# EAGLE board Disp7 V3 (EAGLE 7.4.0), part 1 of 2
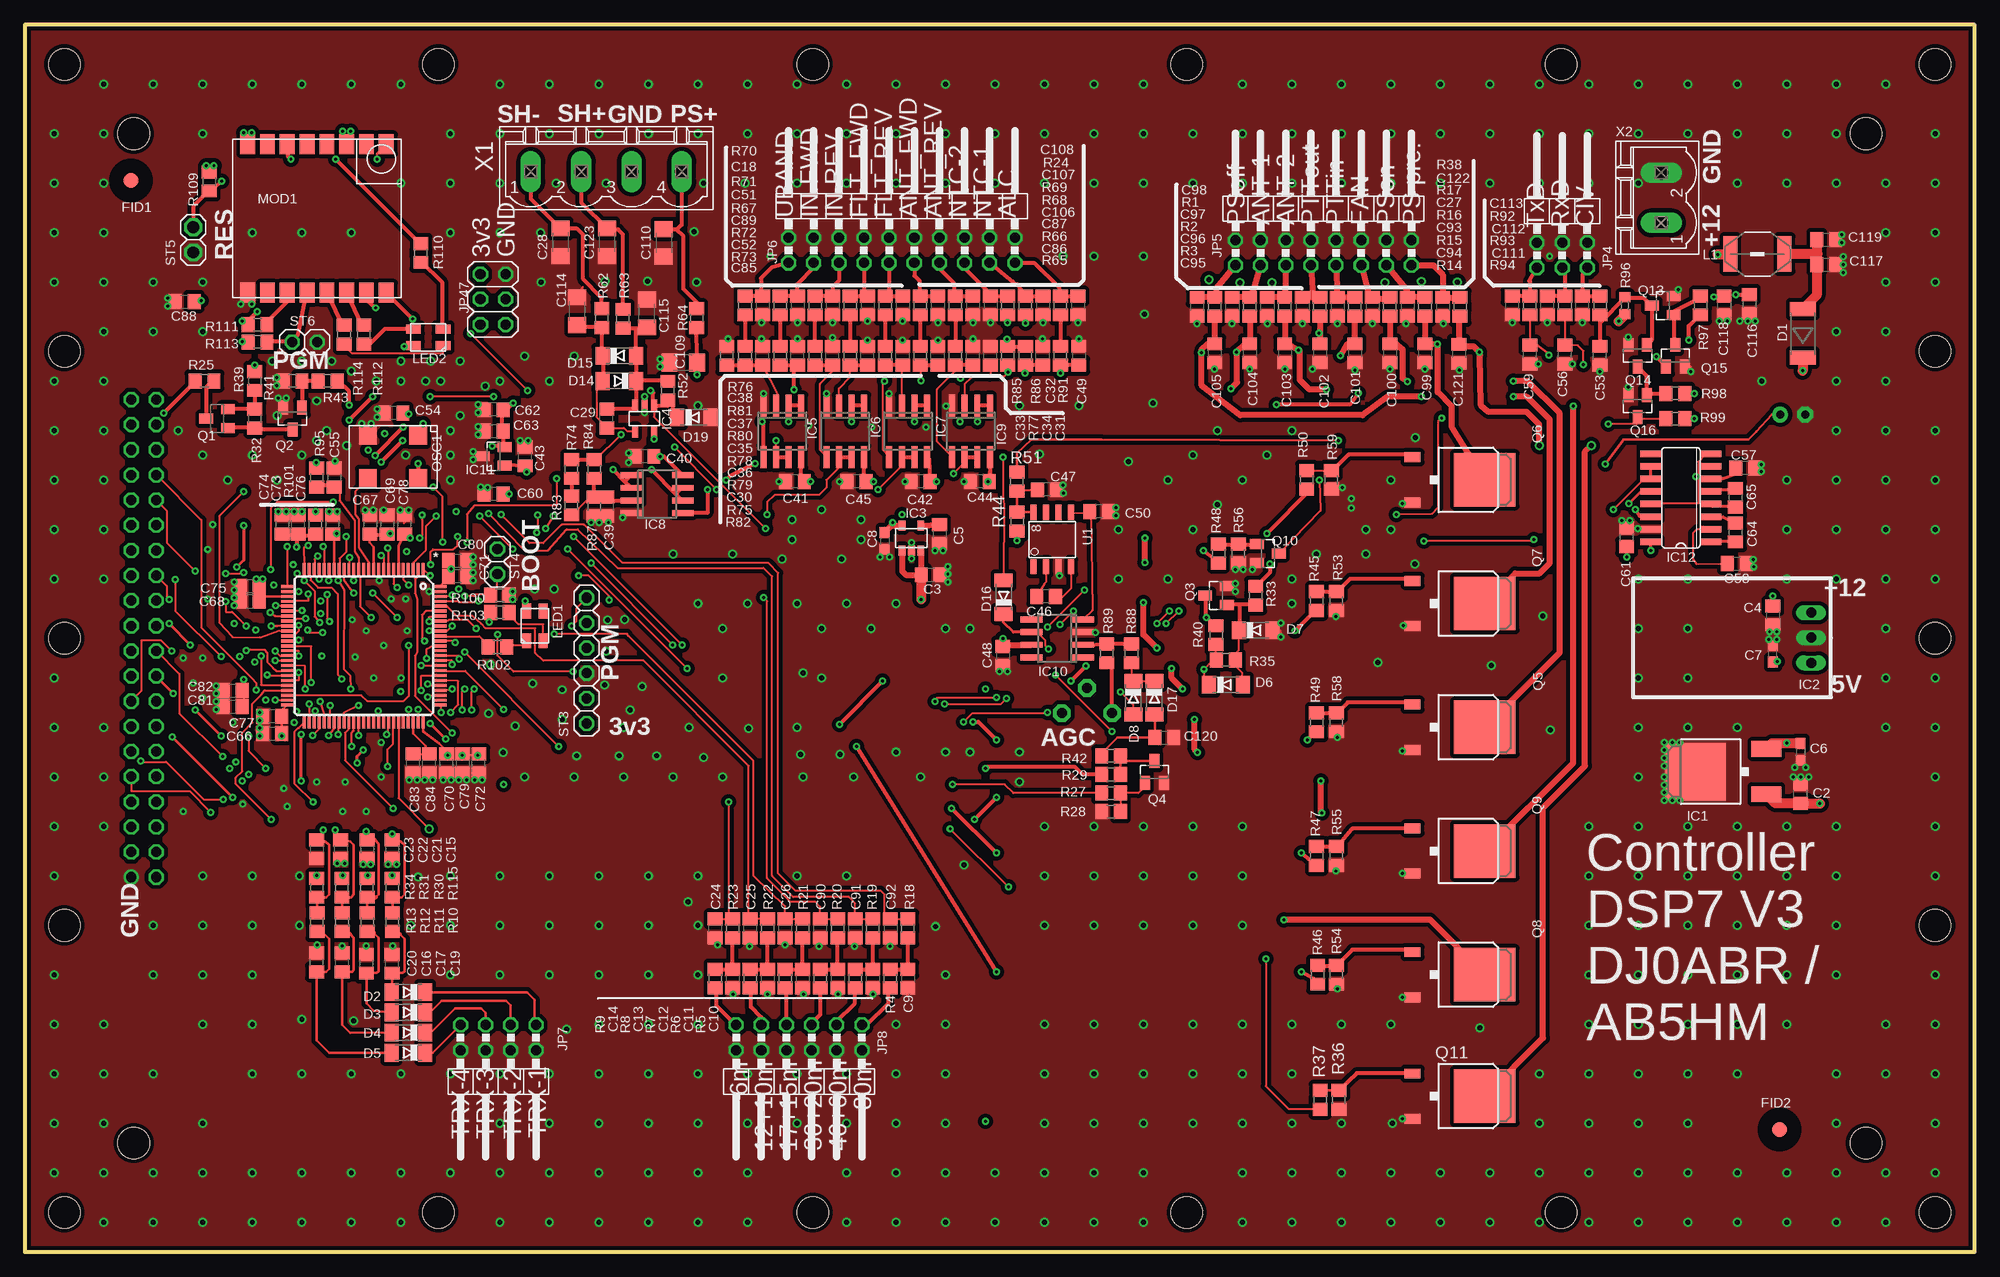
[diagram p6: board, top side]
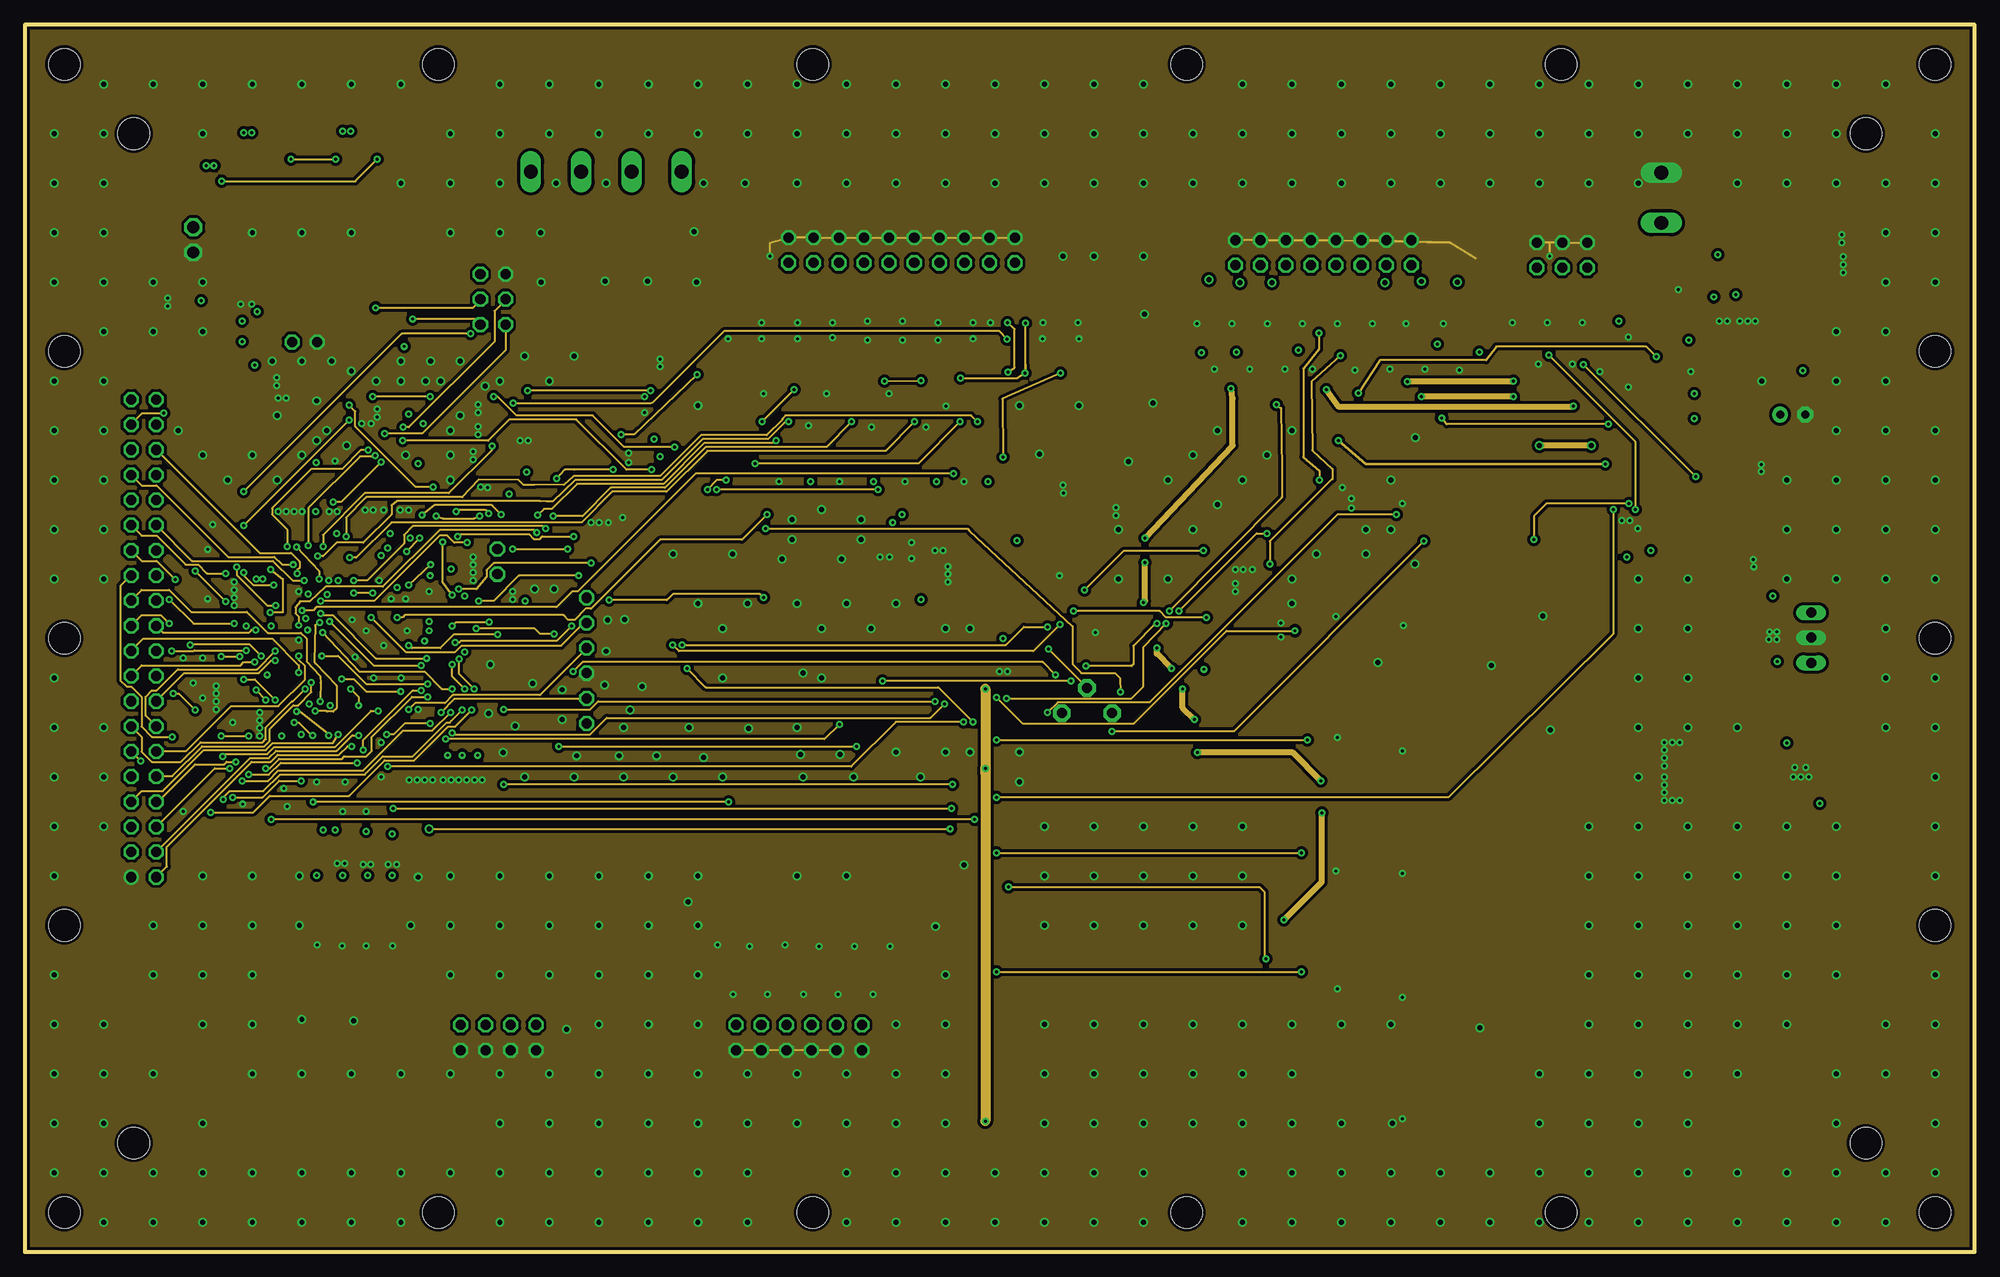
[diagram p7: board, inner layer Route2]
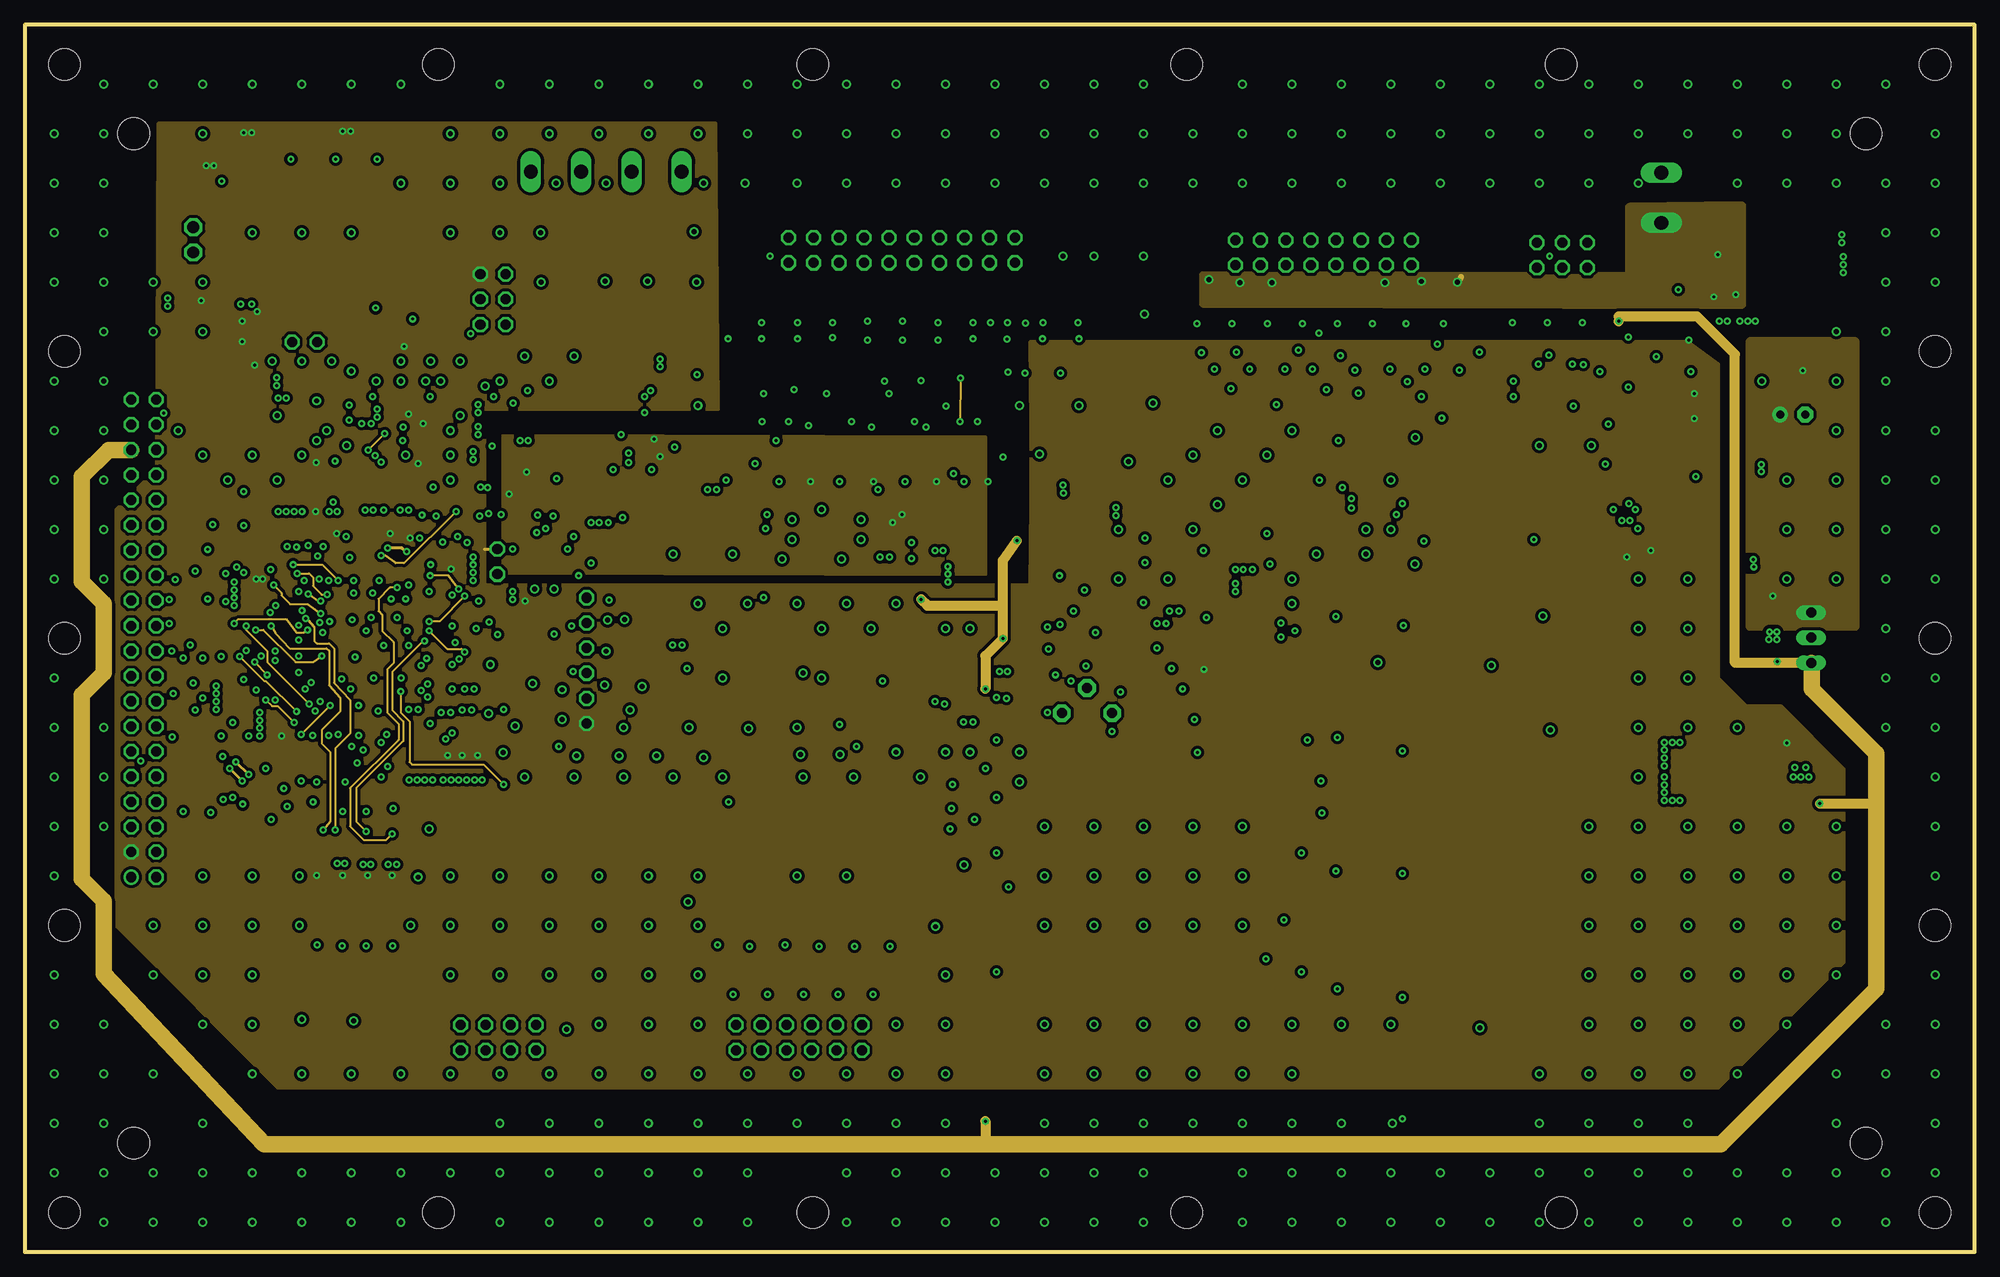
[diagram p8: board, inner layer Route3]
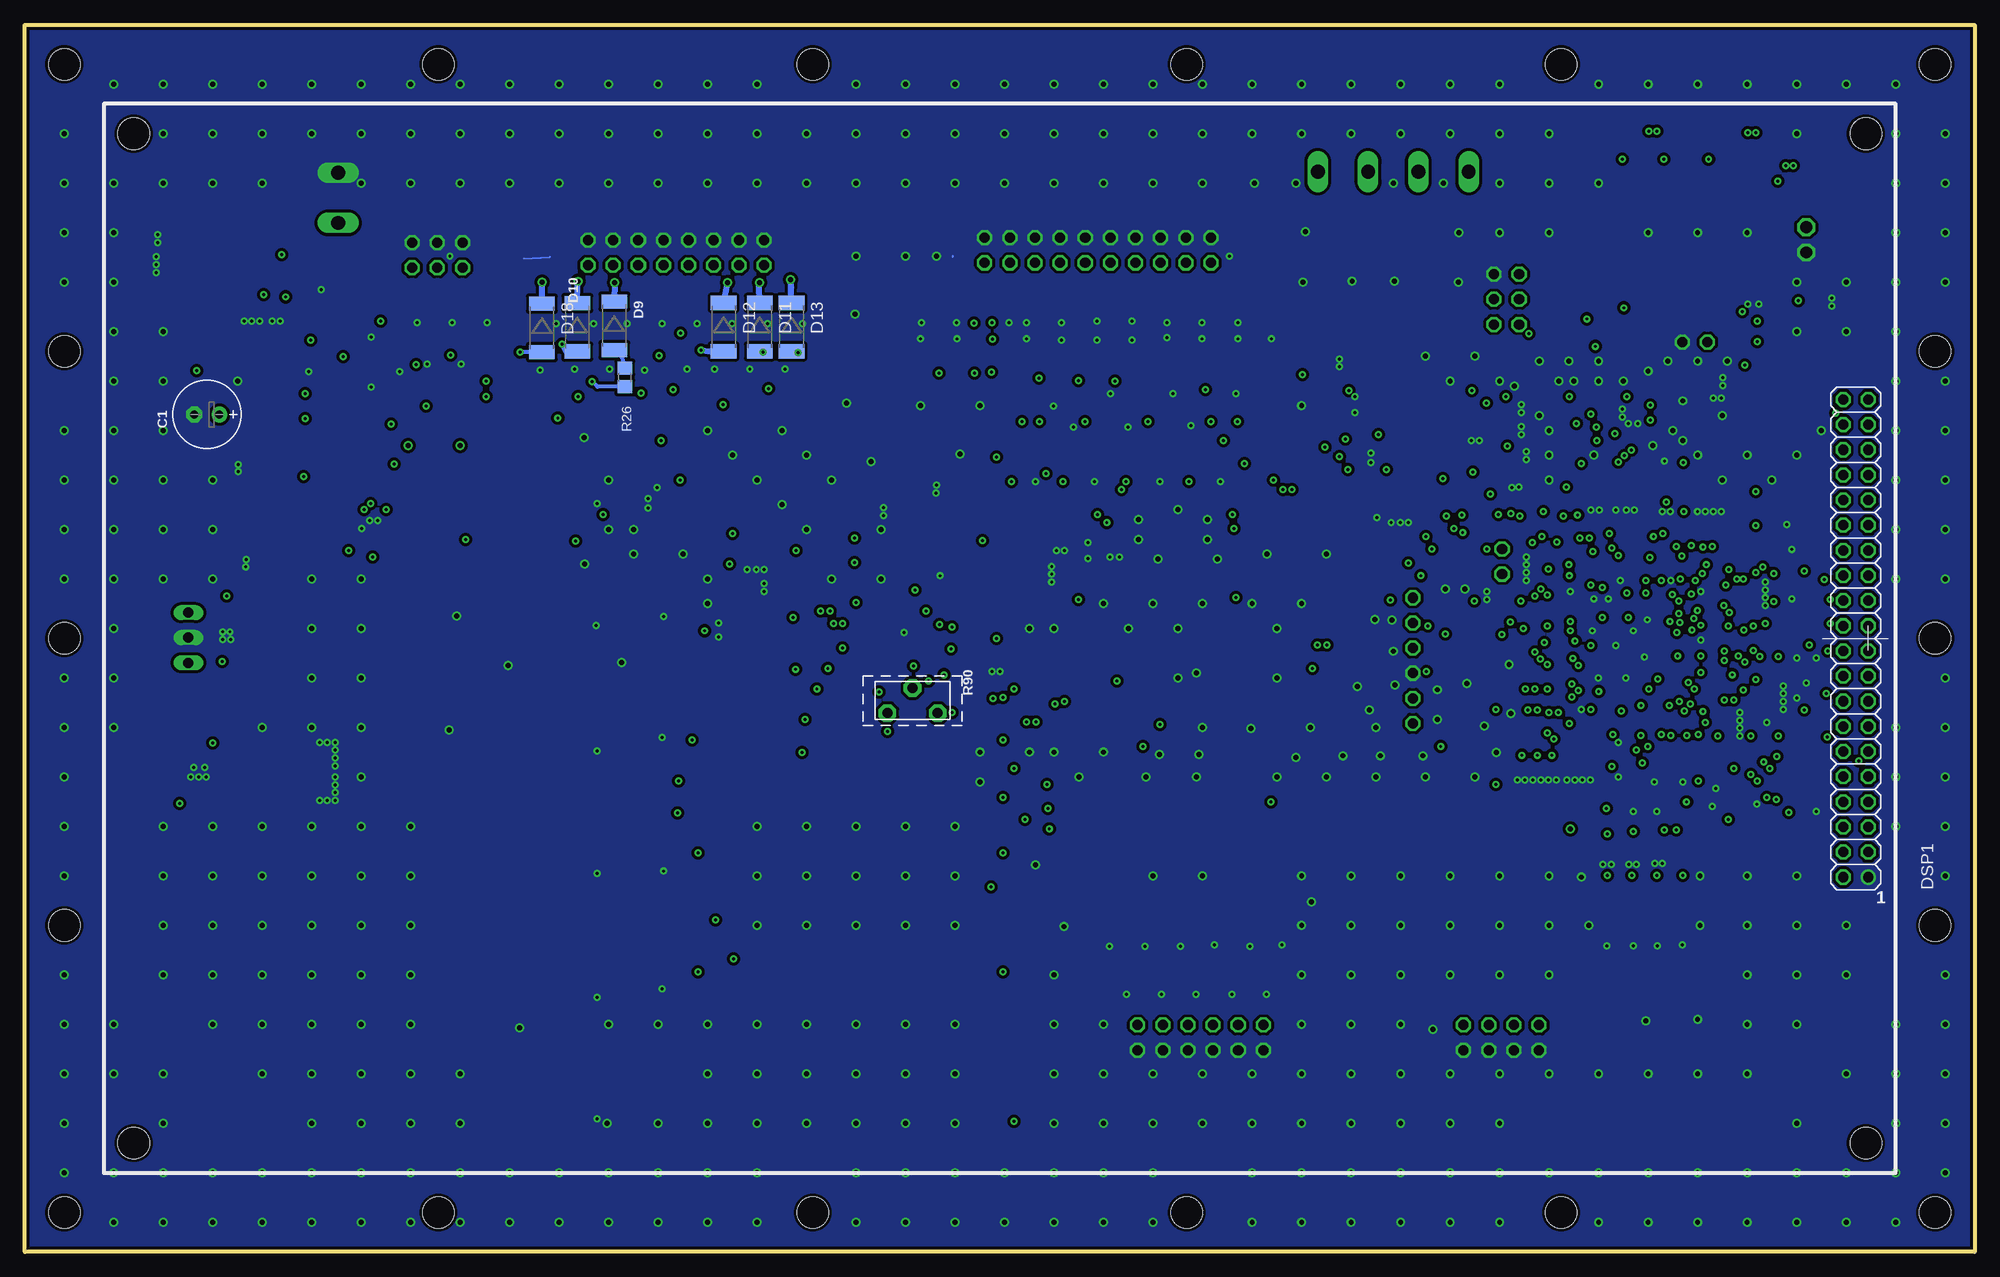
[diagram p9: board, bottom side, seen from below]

Size 197 x 124 mm. Coordinates in mm from the lower left corner, seen from the top.
Outline: 0,0 197,0 197,124 0,124 0,0
Copper layers (1+2*3+16): Top 0.035mm / dielectric 1.5mm / Route2 0.035mm / dielectric 0.15mm / Route3 0.035mm / dielectric 0.2mm / AGND$ 0.035mm
Design rules "default *": minimum track width 8mil, minimum drill 0.3mm, track to track 7mil, track to pad 7mil, pad to pad 7mil, via to via 7mil, smd to smd 0mil, copper to edge 10mil, drill to drill 8mil, minimum pad ring 10mil, minimum via ring 8mil, stop-mask expansion 0.02mm, vias tented up to drill 0.52mm, thermal gap 10mil
Net classes: 0 default: drill 0.3 mm; 1 Supply: width 0.203 mm, drill 0.3 mm, clearance 0.178 mm; 2 v12: drill 0.3 mm; 3 v533: drill 0.3 mm; 4 AGND: width 0.152 mm
Holes 3.2 mm at 4,120 193,120 193,4 4,4 4,91 4,62 4,33 193,91 193,62 193,33 41.8,120 79.6,120 117.4,120 155.2,120 41.8,4 79.6,4 117.4,4 155.2,4

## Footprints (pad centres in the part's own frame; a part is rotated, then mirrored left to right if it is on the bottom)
E2,5-7 = drill 0.813 pad 1.6: + -1.27,0 | drill 0.813 pad 1.6 octagon: - 1.27,0
C0805 = smd 1.3 x 1.5: 1 -0.95,0; 2 0.95,0
C0603 = smd 1.1 x 1: 1 -0.85,0; 2 0.85,0
C1206 = smd 1.6 x 1.8: 1 -1.4,0; 2 1.4,0
MELF = smd 1.45 x 2.6: 1 -2.445,0; 2 2.445,0
MINIMELF = smd 1.4 x 1.8: A 1.7,0; C -1.7,0
2X20 = drill 1.016: 1 2.747,78.13 | drill 1.016 octagon: 2 5.287,78.13; 3 2.747,75.59; 4 5.287,75.59; 5 2.747,73.05; 6 5.287,73.05; 7 2.747,70.51; 8 5.287,70.51; 9 2.747,67.97; 10 5.287,67.97; 11 2.747,65.43; 12 5.287,65.43; 13 2.747,62.89; 14 5.287,62.89; 15 2.747,60.35; 16 5.287,60.35; 17 2.747,57.81; 18 5.287,57.81; 19 2.747,55.27; 20 5.287,55.27; 21 2.747,52.73; 22 5.287,52.73; 23 2.747,50.19; 24 5.287,50.19; 25 2.747,47.65; 26 5.287,47.65; 27 2.747,45.11; 28 5.287,45.11; 29 2.747,42.57; 30 5.287,42.57; 31 2.747,40.03; 32 5.287,40.03; 33 2.747,37.49; 34 5.287,37.49; 35 2.747,34.95; 36 5.287,34.95; 37 2.747,32.41; 38 5.287,32.41; 39 2.747,29.87; 40 5.287,29.87 | hole 3.2: 3,105; 178,105; 178,3; 3,3
FIDUCIAL = smd 1.5 x 1.5: P$1 0,0
DPACK = smd 1.6 x 3: 1 -2.28,-4.8; 3 2.28,-4.8 | smd 5.8 x 6.2: 4 0,2.38
78SR_SWITCHREG = drill 1.016 long: 1 2.54,0; 2 0,0; 3 -2.54,0
SOT23-5 = smd 0.686 x 0.991: 1 -0.953,0; 2 0,0; 3 0.953,0; 4 0.953,2.54; 5 -0.953,2.54
SOT23-5' = smd 0.6 x 1.2: 1 -0.95,-1.306; 2 0,-1.306; 3 0.95,-1.306; 4 0.95,1.306; 5 -0.95,1.306
SO08 = smd 0.6 x 2.2: 1 -1.905,-2.6; 2 -0.635,-2.6; 3 0.635,-2.6; 4 1.905,-2.6; 5 1.905,2.6; 6 0.635,2.6; 7 -0.635,2.6; 8 -1.905,2.6
SOT23@1 = smd 1 x 1.4: 1 -0.95,-1.1; 2 0.95,-1.1; 3 0,1.1
SO16 = smd 0.66 x 2.032: 1 -4.445,-3.073; 2 -3.175,-3.073; 3 -1.905,-3.073; 4 -0.635,-3.073; 5 0.635,-3.073; 6 1.905,-3.073; 7 3.175,-3.073; 8 4.445,-3.073; 9 4.445,3.073; 10 3.175,3.073; 11 1.905,3.073; 12 0.635,3.073; 13 -0.635,3.073; 14 -1.905,3.073; 15 -3.175,3.073; 16 -4.445,3.073
TQFP100 = smd 1.2 x 0.3: 1 -7.75,6; 2 -7.75,5.5; 3 -7.75,5; 4 -7.75,4.5; 5 -7.75,4; 6 -7.75,3.5; 7 -7.75,3; 8 -7.75,2.5; 9 -7.75,2; 10 -7.75,1.5; 11 -7.75,1; 12 -7.75,0.5; 13 -7.75,0; 14 -7.75,-0.5; 15 -7.75,-1; 16 -7.75,-1.5; 17 -7.75,-2; 18 -7.75,-2.5; 19 -7.75,-3; 20 -7.75,-3.5; 21 -7.75,-4; 22 -7.75,-4.5; 23 -7.75,-5; 24 -7.75,-5.5; 25 -7.75,-6; 51 7.75,-6; 52 7.75,-5.5; 53 7.75,-5; 54 7.75,-4.5; 55 7.75,-4; 56 7.75,-3.5; 57 7.75,-3; 58 7.75,-2.5; 59 7.75,-2; 60 7.75,-1.5; 61 7.75,-1; 62 7.75,-0.5; 63 7.75,0; 64 7.75,0.5; 65 7.75,1; 66 7.75,1.5; 67 7.75,2; 68 7.75,2.5; 69 7.75,3; 70 7.75,3.5; 71 7.75,4; 72 7.75,4.5; 73 7.75,5; 74 7.75,5.5; 75 7.75,6 | smd 0.3 x 1.2: 26 -6,-7.75; 27 -5.5,-7.75; 28 -5,-7.75; 29 -4.5,-7.75; 30 -4,-7.75; 31 -3.5,-7.75; 32 -3,-7.75; 33 -2.5,-7.75; 34 -2,-7.75; 35 -1.5,-7.75; 36 -1,-7.75; 37 -0.5,-7.75; 38 0,-7.75; 39 0.5,-7.75; 40 1,-7.75; 41 1.5,-7.75; 42 2,-7.75; 43 2.5,-7.75; 44 3,-7.75; 45 3.5,-7.75; 46 4,-7.75; 47 4.5,-7.75; 48 5,-7.75; 49 5.5,-7.75; 50 6,-7.75; 76 6,7.75; 77 5.5,7.75; 78 5,7.75; 79 4.5,7.75; 80 4,7.75; 81 3.5,7.75; 82 3,7.75; 83 2.5,7.75; 84 2,7.75; 85 1.5,7.75; 86 1,7.75; 87 0.5,7.75; 88 0,7.75; 89 -0.5,7.75; 90 -1,7.75; 91 -1.5,7.75; 92 -2,7.75; 93 -2.5,7.75; 94 -3,7.75; 95 -3.5,7.75; 96 -4,7.75; 97 -4.5,7.75; 98 -5,7.75; 99 -5.5,7.75; 100 -6,7.75
2X03/90 = drill 1.016 octagon: 1 -2.54,-6.35; 2 -2.54,-3.81; 3 0,-6.35; 4 0,-3.81; 5 2.54,-6.35; 6 2.54,-3.81
2X08/90 = drill 1.016 octagon: 1 -8.89,-6.35; 2 -8.89,-3.81; 3 -6.35,-6.35; 4 -6.35,-3.81; 5 -3.81,-6.35; 6 -3.81,-3.81; 7 -1.27,-6.35; 8 -1.27,-3.81; 9 1.27,-6.35; 10 1.27,-3.81; 11 3.81,-6.35; 12 3.81,-3.81; 13 6.35,-6.35; 14 6.35,-3.81; 15 8.89,-6.35; 16 8.89,-3.81
2X10/90 = drill 1.016 octagon: 1 -11.43,-6.35; 2 -11.43,-3.81; 3 -8.89,-6.35; 4 -8.89,-3.81; 5 -6.35,-6.35; 6 -6.35,-3.81; 7 -3.81,-6.35; 8 -3.81,-3.81; 9 -1.27,-6.35; 10 -1.27,-3.81; 11 1.27,-6.35; 12 1.27,-3.81; 13 3.81,-6.35; 14 3.81,-3.81; 15 6.35,-6.35; 16 6.35,-3.81; 17 8.89,-6.35; 18 8.89,-3.81; 19 11.43,-6.35; 20 11.43,-3.81
2X04/90 = drill 1.016 octagon: 1 -3.81,-6.35; 2 -3.81,-3.81; 3 -1.27,-6.35; 4 -1.27,-3.81; 5 1.27,-6.35; 6 1.27,-3.81; 7 3.81,-6.35; 8 3.81,-3.81
2X06/90 = drill 1.016 octagon: 1 -6.35,-6.35; 2 -6.35,-3.81; 3 -3.81,-6.35; 4 -3.81,-3.81; 5 -1.27,-6.35; 6 -1.27,-3.81; 7 1.27,-6.35; 8 1.27,-3.81; 9 3.81,-6.35; 10 3.81,-3.81; 11 6.35,-6.35; 12 6.35,-3.81
2X03 = drill 1.016 octagon: 1 -2.54,-1.27; 2 -2.54,1.27; 3 0,-1.27; 4 0,1.27; 5 2.54,-1.27; 6 2.54,1.27
S = smd 1.4 x 3.56: 1 -2.73,0; 2 2.73,0
PLCC4_WE_LED = smd 1.5 x 0.9: 1 1.51,0.88; 2 1.51,-0.82; 3 -1.49,0.88; 4 -1.49,-0.82
ESP8266-12 = smd 1.5 x 2: P$1 0,0; P$2 2,0; P$3 4,0; P$4 6,0; P$5 8,0; P$6 10,0; P$7 12,0; P$8 14,0; P$9 14,15; P$10 12,15; P$11 10,15; P$12 8,15; P$13 6,15; P$14 4,15; P$15 2,15; P$16 0,15
QOSC_AQO7015 = smd 1.8 x 2: 1 0,-0.318; 2 5.08,-0.318; 3 5.08,4.128; 4 0,4.128
SOT23 = smd 1 x 1.4: 1 -0.95,-1.1; 2 0.95,-1.1; 3 0,1.1
D-PAK_TO252AA = smd 1 x 1.6: 1 -2.28,-4.8; 3 2.28,-4.8 | smd 5.4 x 6.2: 4 0,2.5
R0805 = smd 1.3 x 1.5: 1 -0.95,0; 2 0.95,0
MINIPOTI = drill 1.016 pad 1.778 octagon: 1 -2.54,-2.54; 2 2.54,-2.54; 3 0,0
R0603 = smd 1 x 1.1: 1 -0.85,0; 2 0.85,0
PINHEAD6X1 = drill 1.016 octagon: 1 -6.35,0; 2 -3.81,0; 3 -1.27,0; 4 1.27,0; 5 3.81,0; 6 6.35,0
PINHEAD1X2 = drill 1.016 octagon: 1 -1.27,0; 2 1.27,0
PINHEAD1X2BIG = drill 1.2 octagon: 1 -2.54,0; 2 0,0
SO-8 = smd 0.61 x 1.524: 1 -1.905,-2.743; 2 -0.635,-2.743; 3 0.635,-2.743; 4 1.905,-2.743; 5 1.905,2.743; 6 0.635,2.743; 7 -0.635,2.743; 8 -1.905,2.743
MSTBV4 = drill 1.397 long: 1 -7.62,0; 2 -2.54,0; 3 2.54,0; 4 7.62,0
MSTBV2 = drill 1.397 long: 1 -2.54,0; 2 2.54,0

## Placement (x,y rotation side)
C1  100u/16  [E2,5-7]  178.61,84.63 180 bottom
C2  10u  [C0805]  179.4,46.29 90 top
C3  10u  [C0805]  91.52,68.42 0 top
C4  10u  [C0805]  176.6,64.32 270 top
C5  10n  [C0805]  92.42,72.54 270 top
C6  10u  [C0603]  179.4,50.54 270 top
C7  10u  [C0603]  176.6,60.45 90 top
C8  10u  [C0603]  86.88,71.86 270 top
C9  100n  [C0805]  89.22,27.62 270 top
C10  100n  [C0805]  85.67,27.62 270 top
C11  100n  [C0805]  82.14,27.62 270 top
C12  100n  [C0805]  78.59,27.62 270 top
C13  100n  [C0805]  75.06,27.62 270 top
C14  100n  [C0805]  71.52,27.62 270 top
C15  100n  [C0805]  37.12,40.7 270 top
C16  100n  [C0805]  32.06,29.25 90 top
C17  100n  [C0805]  34.52,29.13 90 top
C18  100n  [C0805]  74.54,95.63 270 top
C19  100n  [C0805]  37.1,29.13 90 top
C20  100n  [C0805]  29.48,29.25 90 top
C21  100n  [C0805]  34.59,40.7 270 top
C22  100n  [C0805]  31.92,40.7 270 top
C23  100n  [C0805]  29.5,40.7 270 top
C24  100n  [C0805]  69.75,32.7 270 top
C25  100n  [C0805]  73.28,32.7 270 top
C26  100n  [C0805]  76.83,32.7 270 top
C27  100n  [C0805]  139.68,95.5 270 top
C28  100n/200V  [C1206]  54.12,102.02 270 top
C29  10u  [C0805]  58.8,84.2 90 top
C30  100n  [C0805]  74.54,90.55 90 top
C31  1u  [C0805]  97.57,90.55 90 top
C32  1u  [C0805]  102.84,90.55 90 top
C33  10n  [C0805]  92.24,90.55 90 top
C34  10n  [C0805]  95.78,90.55 90 top
C35  10n  [C0805]  81.62,90.55 90 top
C36  10n  [C0805]  78.08,90.55 90 top
C37  10n  [C0805]  85.16,90.55 90 top
C38  10n  [C0805]  88.7,90.55 90 top
C39  1u  [C0805]  58.8,75.31 270 top
C40  1u  [C0805]  62.61,80.39 180 top
C41  1u  [C0805]  77.81,77.85 180 top
C42  1u  [C0805]  90.51,77.85 180 top
C43  1u  [C0805]  50.55,80.39 90 top
C44  1u  [C0805]  96.48,77.85 180 top
C45  1u  [C0805]  84.03,77.85 180 top
C46  10u  [C0805]  103.19,66.24 180 top
C47  1u  [C0805]  103.27,77.02 180 top
C48  1u  [C0805]  98.81,60.24 270 top
C49  10n  [C0805]  106.48,90.55 270 top
C50  10u  [C0805]  108.54,74.81 180 top
C51  10n  [C0805]  78.08,95.63 270 top
C52  10n  [C0805]  85.16,95.63 270 top
C53  1n  [C0805]  159.13,90.55 90 top
C54  1u  [C0805]  37.25,84.75 180 top
C55  100n  [C0805]  31.25,78.25 270 top
C56  1n  [C0805]  155.59,90.67 90 top
C57  1u  [C0805]  173.82,79.21 180 top
C58  1u  [C0805]  172.96,69.56 0 top
C59  1n  [C0805]  152.05,90.67 90 top
C60  100n  [C0805]  47.37,76.58 180 top
C61  1u  [C0805]  161.82,72.21 270 top
C62  100n  [C0805]  47.37,85.09 180 top
C63  1u  [C0805]  47.37,82.93 0 top
C64  1u  [C0805]  172.82,72.71 270 top
C65  1u  [C0805]  172.82,76.21 270 top
C66  4u7  [C0805]  25,52.38 0 top
C67  100n  [C0805]  34.88,73.5 270 top
C68  100n  [C0805]  22.75,65.75 0 top
C69  100n  [C0805]  36.62,73.5 270 top
C70  100n  [C0805]  42.62,49.38 90 top
C71  100n  [C0805]  43.75,68.25 180 top
C72  100n  [C0805]  45.88,49.38 90 top
C73  100n  [C0805]  27.62,73.5 90 top
C74  1u  [C0805]  26,73.5 270 top
C75  100n  [C0805]  22.75,67.25 180 top
C76  100n  [C0805]  31.12,73.5 90 top
C77  100n  [C0805]  25,54.12 180 top
C78  100n  [C0805]  38.38,73.5 90 top
C79  100n  [C0805]  44.25,49.38 270 top
C80  100n  [C0805]  43.75,69.88 0 top
C81  1u  [C0805]  21,55.12 0 top
C82  1u  [C0805]  21,56.75 0 top
C83  1u  [C0805]  39.25,49.38 90 top
C84  1u  [C0805]  40.88,49.38 90 top
C85  10n  [C0805]  88.7,95.63 270 top
C86  10n  [C0805]  92.24,95.63 270 top
C87  10n  [C0805]  95.78,95.63 270 top
C88  10u  [C0805]  16.16,96.04 0 top
C89  10n  [C0805]  81.62,95.63 270 top
C90  100n  [C0805]  80.36,32.7 270 top
C91  100n  [C0805]  83.91,32.7 270 top
C92  100n  [C0805]  87.44,32.7 270 top
C93  100n  [C0805]  136.14,95.5 270 top
C94  100n  [C0805]  132.6,95.5 270 top
C95  100n  [C0805]  129.06,95.5 270 top
C96  100n  [C0805]  125.52,95.5 270 top
C97  100n  [C0805]  121.98,95.5 270 top
C98  100n  [C0805]  118.44,95.5 270 top
C99  100n  [C0805]  141.45,90.8 270 top
C100  100n  [C0805]  137.91,90.8 270 top
C101  100n  [C0805]  134.37,90.8 270 top
C102  100n  [C0805]  130.83,90.8 270 top
C103  100n  [C0805]  127.29,90.8 270 top
C104  100n  [C0805]  123.75,90.8 270 top
C105  100n  [C0805]  120.21,90.8 270 top
C106  100n  [C0805]  97.57,95.63 270 top
C107  100n  [C0805]  102.86,95.63 270 top
C108  100n  [C0805]  106.4,95.63 270 top
C109  100n/200V  [C1206]  66.52,89.85 180 top
C110  100n/200V  [C1206]  64.55,101.95 270 top
C111  1n  [C0805]  157.36,95.63 90 top
C112  1n  [C0805]  153.82,95.63 90 top
C113  1n  [C0805]  150.28,95.63 90 top
C114  100n/200V  [C1206]  55.81,95.06 90 top
C115  100n/200V  [C1206]  62.87,94.82 90 top
C116  10u  [C0805]  174.21,95.79 270 top
C117  10u  [C0805]  181.99,99.76 0 top
C118  100n  [C0805]  171.67,95.63 270 top
C119  100n  [C0805]  181.99,102.3 0 top
C120  10n  [C0805]  115.12,52 0 top
C121  100n  [C0805]  144.88,90.75 270 top
C122  100n  [C0805]  143.25,95.5 270 top
C123  100n/200V  [C1206]  58.83,102.03 270 top
D1  1N4001  [MELF]  179.62,92.81 90 top
D2  1N4448  [MINIMELF]  38.76,26.25 180 top
D3  1N4448  [MINIMELF]  38.76,24.21 180 top
D4  1N4448  [MINIMELF]  38.76,22.17 180 top
D5  1N4448  [MINIMELF]  38.76,20.13 180 top
D6  NTS245SFT1G  [MINIMELF]  121.35,57.32 0 top
D7  NTS245SFT1G  [MINIMELF]  124.35,62.82 0 top
D8  1N4448  [MINIMELF]  112,56 270 top
D9  SS110B  [MELF]  137.44,93.58 270 bottom
D10  SS110B  [MELF]  141.18,93.43 270 bottom
D11  SS110B  [MELF]  122.75,93.45 270 bottom
D12  SS110B  [MELF]  126.39,93.45 270 bottom
D13  SS110B  [MELF]  119.54,93.45 270 bottom
D14  NTS245SFT1G  [MINIMELF]  60.07,88.01 180 top
D15  NTS245SFT1G  [MINIMELF]  60.07,90.55 0 top
D16  1N4448  [MINIMELF]  98.88,66.16 90 top
D17  1N4448  [MINIMELF]  114.12,56 270 top
D18  SS110B  [MELF]  144.75,93.38 270 bottom
D19  *3V  [MINIMELF]  67.6,84.33 0 top
DSP1  DISPLAY7DISPL7_ARDUINO  [2X20]  8,116 180 bottom
FID1  FIDUCIAL  [FIDUCIAL]  10.73,108.26 0 top
FID2  FIDUCIAL  [FIDUCIAL]  177.29,12.37 0 top
IC1  LF33CDT-DPAK  [DPACK]  171.15,48.54 90 top
IC2  7805 (7962138)  [78SR_SWITCHREG]  180.48,62.07 90 top
IC3  LP2992 3v3  [SOT23-5]  89.58,70.87 0 top
IC4  INA193AQDBVRQ1  [SOT23-5']  62.61,84.2 180 top
IC5  TS27L2C  [SO08]  76.54,82.93 180 top
IC6  TS27L2C  [SO08]  82.89,82.93 180 top
IC7  TS27L2C  [SO08]  89.24,82.93 180 top
IC8  TS27L2C  [SO08]  63.88,76.58 270 top
IC9  TS27L2C  [SO08]  95.59,82.93 180 top
IC10  TL081D  [SO08]  104.31,61.99 90 top
IC11  ADR381  [SOT23@1]  47.37,80.39 90 top
IC12  MAX3232  [SO16]  167.32,76.21 90 top
IC13  STM32F427VGT6  [TQFP100]  34.25,61.25 270 top
JP4  [2X03/90]  155.32,105.79 0 top
JP5  [2X08/90]  131.2,106.04 0 top
JP6  [2X10/90]  88.59,106.29 0 top
JP7  TRX Detector  [2X04/90]  47.84,16.59 180 top
JP8  Band Relais  [2X06/90]  78.22,16.59 180 top
JP47  [2X03]  47.3,96.26 270 top
L1  WE74451147/47uH  [S]  175.05,100.84 180 top
LED1  RGBLED  [PLCC4_WE_LED]  51.57,63.25 90 top
LED2  RGBLED  [PLCC4_WE_LED]  40.77,92.44 180 top
MOD1  ESP-07S (ESP8266)  [ESP8266-12]  22.52,96.94 0 top
OSC1  OSZ8MHz  [QOSC_AQO7015]  39.75,82.25 180 top
Q1  IRLML6401  [SOT23]  19.43,84.2 90 top
Q2  N-CH_MOSFET  [SOT23]  27.05,84.2 180 top
Q3  N-CH_MOSFET  [SOT23]  120.35,66.32 90 top
Q4  BS170_SMD  [SOT23]  114.12,48.5 0 top
Q5  IRLR120N  [D-PAK_TO252AA]  145,53.02 270 top
Q6  IRLR120N  [D-PAK_TO252AA]  145,78.02 270 top
Q7  IRLR120N  [D-PAK_TO252AA]  145,65.52 270 top
Q8  IRLR120N  [D-PAK_TO252AA]  145,28.02 270 top
Q9  IRLR120N  [D-PAK_TO252AA]  145,40.52 270 top
Q10  N-CH_MOSFET  [SOT23]  125.6,70.57 270 top
Q11  IRLR120N  [D-PAK_TO252AA]  145,15.75 270 top
Q13  N-CH_MOSFET  [SOT23]  165.48,95.63 90 top
Q14  N-CH_MOSFET  [SOT23]  162.94,90.55 180 top
Q15  N-CH_MOSFET  [SOT23]  166.75,90.55 0 top
Q16  N-CH_MOSFET  [SOT23]  162.94,85.47 180 top
R1  1kOhm-Ferrit  [R0805]  120.21,95.5 270 top
R2  1kOhm-Ferrit  [R0805]  123.75,95.5 270 top
R3  1kOhm-Ferrit  [R0805]  127.29,95.5 270 top
R4  100  [R0805]  87.44,27.62 90 top
R5  100  [R0805]  83.91,27.62 90 top
R6  100  [R0805]  80.36,27.62 90 top
R7  100  [R0805]  76.83,27.62 90 top
R8  100  [R0805]  73.28,27.62 90 top
R9  100  [R0805]  69.75,27.62 90 top
R10  1kOhm-Ferrit  [R0805]  37.15,33.33 90 top
R11  1kOhm-Ferrit  [R0805]  34.61,33.33 90 top
R12  1kOhm-Ferrit  [R0805]  32.06,33.33 90 top
R13  1kOhm-Ferrit  [R0805]  29.52,33.33 90 top
R14  1kOhm-Ferrit  [R0805]  130.83,95.5 270 top
R15  1kOhm-Ferrit  [R0805]  134.37,95.5 270 top
R16  1kOhm-Ferrit  [R0805]  137.91,95.5 270 top
R17  1kOhm-Ferrit  [R0805]  141.45,95.5 270 top
R18  1kOhm-Ferrit  [R0805]  89.22,32.7 270 top
R19  1kOhm-Ferrit  [R0805]  85.67,32.7 270 top
R20  1kOhm-Ferrit  [R0805]  82.14,32.7 270 top
R21  1kOhm-Ferrit  [R0805]  78.59,32.7 270 top
R22  1kOhm-Ferrit  [R0805]  75.06,32.7 270 top
R23  1kOhm-Ferrit  [R0805]  71.52,32.7 270 top
R24  1kOhm-Ferrit  [R0805]  104.63,95.63 90 top
R25  220  [R0805]  18.16,88.01 0 top
R26  ***  [R0805]  136.38,88.38 270 bottom
R27  1k  [R0805]  109.75,46.38 0 top
R28  100k  [R0805]  109.75,44.5 0 top
R29  1k  [R0805]  109.75,48.25 180 top
R30  10k  [R0805]  34.59,36.8 90 top
R31  10k  [R0805]  32.05,36.8 90 top
R32  1k  [R0805]  23.24,84.2 270 top
R33  1k  [R0805]  124.35,66.32 270 top
R34  10k  [R0805]  29.5,36.8 90 top
R35  1M  [R0805]  121.35,59.82 0 top
R36  100k  [R0805]  132.75,15.38 270 top
R37  1k  [R0805]  130.88,15.38 90 top
R38  1kOhm-Ferrit  [R0805]  145,95.5 270 top
R39  100  [R0805]  23.24,88.01 90 top
R40  100k  [R0805]  120.35,62.32 270 top
R41  100k  [R0805]  27.05,88.01 180 top
R42  10k  [R0805]  109.75,50.12 0 top
R43  1k  [R0805]  30.61,88.01 180 top
R44  oR  [R0805]  100.25,73.8 90 top
R45  1k  [R0805]  130.5,65.77 90 top
R46  1k  [R0805]  130.62,28.02 90 top
R47  1k  [R0805]  130.5,40.02 90 top
R48  1k  [R0805]  120.6,70.57 90 top
R49  1k  [R0805]  130.5,53.52 90 top
R50  1k  [R0805]  129.5,78.02 90 top
R51  ***  [R0805]  100.22,77.85 270 top
R52  *10k  [R0805]  64.97,87.03 270 top
R53  100k  [R0805]  132.5,65.77 270 top
R54  100k  [R0805]  132.5,28.02 270 top
R55  100k  [R0805]  132.5,40.02 270 top
R56  100k  [R0805]  122.6,70.57 270 top
R58  100k  [R0805]  132.5,53.52 270 top
R59  100k  [R0805]  132,78.02 270 top
R62  1kOhm-Ferrit  [R0805]  58.3,94.36 270 top
R63  1kOhm-Ferrit  [R0805]  60.44,94.28 270 top
R64  1kOhm-Ferrit  [R0805]  67.88,94.36 270 top
R65  1kOhm-Ferrit  [R0805]  90.47,95.63 270 top
R66  1kOhm-Ferrit  [R0805]  94.01,95.63 270 top
R67  1kOhm-Ferrit  [R0805]  79.85,95.63 270 top
R68  1kOhm-Ferrit  [R0805]  99.3,95.63 270 top
R69  1kOhm-Ferrit  [R0805]  101.09,95.63 270 top
R70  1kOhm-Ferrit  [R0805]  72.77,95.63 270 top
R71  1kOhm-Ferrit  [R0805]  76.31,95.63 270 top
R72  1kOhm-Ferrit  [R0805]  83.39,95.63 270 top
R73  1kOhm-Ferrit  [R0805]  86.93,95.63 270 top
R74  NC  [R0805]  55.24,79.12 90 top
R75  22k  [R0805]  72.77,90.55 90 top
R76  1k  [R0805]  90.47,90.55 90 top
R77  1k  [R0805]  94.01,90.55 90 top
R78  1k  [R0805]  79.85,90.55 90 top
R79  1k  [R0805]  76.31,90.55 90 top
R80  1k  [R0805]  83.39,90.55 90 top
R81  1k  [R0805]  86.93,90.55 90 top
R82  10k  [R0805]  70.93,90.55 270 top
R83  390k/0,1%  [R0805]  55.24,75.44 90 top
R84  390k/0,1%  [R0805]  57.53,79.12 90 top
R85  8k2  [R0805]  99.3,90.55 270 top
R86  8k2  [R0805]  101.09,90.55 270 top
R87  10k/0,1%  [R0805]  57.53,75.31 90 top
R88  10k  [R0805]  111.81,60.49 90 top
R89  1k  [R0805]  109.31,60.49 90 top
R90  50k  [MINIPOTI]  107.31,56.99 0 bottom
R91  100  [R0805]  104.63,90.55 90 top
R92  1kOhm-Ferrit  [R0805]  152.05,95.63 270 top
R93  1kOhm-Ferrit  [R0805]  155.59,95.63 270 top
R94  1kOhm-Ferrit  [R0805]  159.13,95.63 270 top
R95  100k  [R0805]  29.5,78.25 270 top
R96  10k  [R0603]  161.67,95.63 270 top
R97  10k  [R0805]  169.29,95.63 270 top
R98  10k  [R0805]  166.75,86.74 0 top
R99  10k  [R0805]  166.75,84.2 0 top
R100  10k  [R0805]  48,66.38 180 top
R101  1kOhm-Ferrit  [R0805]  29.38,73.5 270 top
R102  2k2  [R0805]  47.75,61.12 180 top
R103  680  [R0805]  48,64.62 180 top
R109  100k  [R0805]  18.64,108.16 90 top
R110  1k  [R0805]  40.02,100.94 90 top
R111  100k  [R0805]  23.52,93.69 180 top
R112  1k  [R0805]  34.27,92.69 90 top
R113  100k  [R0805]  23.52,91.94 180 top
R114  1k  [R0805]  32.27,92.69 90 top
R115  10k  [R0805]  37.12,36.8 90 top
ST3  SWD  [PINHEAD6X1]  56.75,59.75 90 top
ST4  [PINHEAD1X2]  47.75,69.75 270 top
ST5  [PINHEAD1X2BIG]  17.03,103.54 90 top
ST6  PGM  [PINHEAD1X2]  28.27,91.94 180 top
U1  TC7662AEPASOIC  [SO-8]  103.81,71.99 0 top
X1  MSTBV4  [MSTBV4]  58.75,109.15 0 top
X2  MSTBV2  [MSTBV2]  165.32,106.53 90 top

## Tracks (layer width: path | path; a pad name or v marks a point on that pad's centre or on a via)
+5V  (via drill 0.3)
  Top 0.203: 176.45,59.7 C7.1 | v98.81,61.98 98.96,61.82 98.96,61.66 99.08,61.35
  Top 0.254: 100.27,72.83 R44.1 v100.22,71.88
  Top 0.305: v177.04,59.66 176.45,59.7
  Top 0.406: R29.2 106.88,48.25 106.12,49 97.18,49 v97.06,48.88
  Top 0.61: IC3.3 90.57,70.83 C3.1 89.02,68.42 88.64,68.8 88.64,70.85 IC3.1 | 98.81,61.09 C48.1 99.08,61.35 IC10.7
  Top 1.016: IC1.1 176.87,45.34 C2.1 179.43,45.31 v181.35,45.31 | v161.03,94.04 161.67,94.68 R96.2 | C3.1 90.55,68.41 v90.55,65.94
  Route2 0.406: 97.06,13.24 97,13.24 v97.08,13.22
  Route2 1.016: v97.06,56.9 v97.06,48.88 | 97.06,48.38 v97.06,48.88 | v97.06,48.88 97.06,13.24
  Route3 0.406: v97.08,13.22 97.06,13.22 | v177.04,59.66 180.48,59.66 IC2.3
  Route3 1.016: IC2.3 172.78,59.53 172.78,90.71 168.97,94.52 161.03,94.52 v161.03,94.04 | 98.81,65.31 v98.81,61.98 97.06,60.23 v97.06,56.9 | 98.81,65.31 98.81,69.88 v100.22,71.88 | v181.35,45.31 187.07,45.31 | v90.55,65.94 91.19,65.31 98.81,65.31 | 97.06,13.24 97.06,13.22 97.06,10.86
  Route3 1.676: IC2.3 180.56,59.45 180.56,56.9 187.07,50.39 187.07,45.31 187.07,26.57 171.35,10.86 97.06,10.86 24.19,10.86 8,28.08 8,35.46 5.78,37.69 5.78,56.26 8,58.48 8,65.5 5.78,67.72 5.78,78.33 8.5,81.05 DSP1.35
+UB  (via drill 0.3)
  Top 0.203: 176.58,65.32 C4.1 | 179.61,90.31 D1.1
  Top 0.254: v159.7,79.6 161.43,82 161.5,82.08 174.1,82.08 174.93,82.9 176.5,84.62 C1.+ | v132.7,82 108.78,82.08 101.72,82.08 100.22,80.72 R51.1
  Top 0.305: v176.58,66.26 176.58,65.32
  Top 1.016: 179.61,90.31 v179.61,89.04
  Route2 0.254: v159.7,79.6 135.47,79.6 v132.7,82
  pour Route3 (isolate 0.305, no thermals): 174.37,91.98 184.85,91.98 184.85,63.24 174.37,63.24
/CS  (via drill 0.3)
  Top 0.203: v40.62,59.99 40.62,60.93 41.26,61.26 IC13.88 | v22.13,68.64 21.81,68.64 21.73,68.56 v20.3,68.56
  Route2 0.203: v40.62,59.99 35.46,59.99 31.1,64.36 30.15,64.36 v29.91,64.49 | v25.14,67.37 23.08,67.37 22.13,68.33 v22.13,68.64 | v20.3,68.56 18.4,68.56 17.52,69.44 16.26,69.44 13.32,72.37 11.81,72.37 10.78,73.41 DSP1.29
  Route3 0.203: v29.91,64.49 28.56,65.47 26.81,65.47 25.94,66.34 25.94,66.58 v25.14,67.37
/RD  (via drill 0.3)
  Top 0.203: v43.16,59.36 43.16,59.75 42.05,59.75 IC13.85 | v44.43,56.9 44.2,56.66 v44.2,54.75 | v20.07,45.7 18.08,45.7 14.27,49.51 11.73,49.51 v11.73,49.59
  Route2 0.203: v43.16,59.36 43.16,58.16 v44.43,56.9 | v44.2,54.75 42.92,53.48 42.61,53.48 39.19,50.07 36.18,50.07 34.35,48.24 25.78,48.24 24.11,46.58 20.7,46.58 20.07,45.94 v20.07,45.7 | v11.73,49.59 10.78,50.55 DSP1.11
/RES  (via drill 0.3)
  Top 0.203: v33.71,55.22 32.25,54.5 32.21,54.46 32.21,53.56 IC13.59 | v31.65,67.85 32.25,66.88 32.22,58.9 32.88,58.25 v32.9,56.9
  Route2 0.203: v33.71,55.22 33.71,56.1 v32.9,56.9 | v27.13,69.44 26.02,69.44 25.22,70.23 20.54,70.23 13.32,77.45 11.81,77.45 10.78,78.48 DSP1.33
  Route3 0.203: v31.65,67.85 30.07,69.44 v27.13,69.44
/RW  (via drill 0.3)
  Top 0.203: v43.88,59.91 43.88,60.23 42.05,60.23 IC13.86 | v45.39,56.9 45.15,56.66 v45.15,54.75 | v18.8,44.43 16.65,46.58 10.78,46.58 10.78,48.01 DSP1.9
  Route2 0.203: v43.88,59.91 43.88,58.4 v45.39,56.9 | v45.15,54.75 43.48,53.09 42.77,53.09 39.35,49.67 36.34,49.67 32.77,46.1 24.75,46.1 23.08,44.43 v18.8,44.43
AGC  (via drill 0.3)
  Top 0.203: IC13.24 28.75,68.38 28.88,68.12 28.88,67.88 29.62,67.12 31,67.12 31.62,66.5 31.62,58.38 v32,57.88 | R27.1 99.88,46.38 99,47.25 v93.75,47.25
  Route2 0.203: v93.75,47.25 v48.38,47.25 | v32,57.88 33.25,57.88 34.5,56.62 v38,56.62
  Route3 0.203: v38,56.62 38,54.5 38.88,53.62 38.88,49.5 39.12,49.25 46.38,49.25 v48.38,47.25
AGND  (via drill 0.3, 0.5)
  Top 0.203: v19.34,55.62 19.59,55.31 20.3,55.31 C81.1 | v19.34,56.42 19.34,56.74 20.3,56.74 C82.1 | v35.62,84.36 35.62,84.68 36.34,84.68 C54.2 | v39.63,47.69 39.25,48.21 39.02,48.45 C83.1 | v41.22,47.69 40.84,48.13 40.52,48.45 C84.1 | v174.66,69.23 173.79,69.21 173.85,69.27 C58.2 | v175.45,79.58 175.2,79.27 174.89,79.27 C57.1 | v23.72,52.93 23.84,52.89 24.35,52.77 C66.1 | v23.72,54.51 23.72,54.28 24.35,54.28 C77.2 | v42.26,47.69 42.51,48.01 41.95,48.45 C70.1 | v21.18,66.1 21.18,65.78 21.89,65.78 C68.1 | v43.85,47.69 43.97,48.21 44.09,48.32 C79.2 | v21.18,66.9 21.18,67.21 21.89,67.21 C75.2 | v45.44,47.69 45.31,48.29 45.22,48.45 C72.1 | v26.41,74.83 26.41,74.28 26.26,74.12 C74.1 | v28,74.83 28,74.36 27.76,74.12 C73.2 | v30.76,74.83 30.76,74.44 30.7,74.12 C76.2 | v31.34,79.91 31.34,79.2 31.26,79.12 C55.1 | v35.2,74.96 34.83,74.12 C67.1 | v38.76,74.98 38.64,73.96 38.32,73.64 C78.2 | v49.27,65.94 49.27,66.18 48.64,66.18 R100.1 | v45.31,68.64 45.31,68.33 44.67,68.33 C71.1 | R41.2 25.46,88.01 v25.46,88.33 | v45.31,69.44 45.31,69.67 44.67,69.67 C80.2 | C60.2 45.78,76.58 v46.03,77.27 | C63.1 45.78,82.93 v45.78,82.61 | v50.86,81.98 50.86,81.58 50.55,81.26 C43.2 | C62.2 45.78,85.47 v45.78,85.63 | v57.21,73.72 57.21,74.12 57.53,74.44 R87.1 | v58.96,73.72 58.96,74.28 58.8,74.44 C39.2 | C40.2 61.02,80.39 v61.02,80.71 | v76.22,77.85 C41.2 | v82.32,77.85 C45.2 | v98.49,58.64 98.49,59.04 98.81,59.36 C48.2 | v86.42,70.23 86.42,70.55 86.82,70.94 C8.2 | v71.06,92.26 R82.1 | v132.62,26.57 132.62,27.05 132.54,27.13 R54.2 | C5.2 92.77,71.34 v92.77,70.86 | v74.42,92.26 C30.2 | v88.92,77.85 C42.2 | v78.08,92.26 C36.2 | v74.42,93.92 C18.2
  Top 0.203: v81.62,92.39 C35.2 | v94.9,77.85 C44.2 | v78.08,93.92 C51.2 | v132.46,38.48 132.46,39.12 R55.2 | v85.16,92.14 C37.2 | v81.62,93.92 C89.2 | v88.7,92.14 C38.2 | v85.16,94.04 C52.2 | 104.27,76.93 104.51,77.4 v104.89,77.5 | v92.24,92.14 C33.2 | v88.7,94.04 C85.2 | v95.78,92.26 C34.2 | v92.24,93.92 C86.2 | v95.78,93.92 C87.2 | v106.48,92.26 C49.1 | v132.62,51.97 132.62,52.53 132.54,52.61 R58.2 | v102.86,93.92 C107.2 | v106.4,93.92 C108.2 | v122.3,68.96 122.3,69.44 122.54,69.67 R56.2 | v37.15,30.91 C19.2 | v132.46,64.2 132.46,64.91 R53.2 | v34.48,30.91 C17.2 | v32.06,30.91 C16.2 | v87.43,30.89 C92.2 | v29.52,31.03 C20.2 | v83.84,30.89 C91.2 | 89.16,25.84 C9.2 | v133.09,77.22 132.06,77.22 R59.2 | v80.26,30.89 C90.2 | v76.8,31.01 C26.2 | v73.22,30.89 C25.2 | v70,31.01 C24.2 | v120.21,89.21 C105.2 | v123.75,89.21 C104.2 | v118.44,93.79 C98.2 | v127.29,89.21 C103.2 | v121.98,93.79 C97.2 | v179.93,48.96 179.93,49.2 179.45,49.67 C6.2 | v130.08,89.21 C102.2 | v125.52,93.79 C96.2 | v134.37,89.09 C101.2 | v129.06,93.79 C95.2 | v162.15,73.88 162.15,73.41 161.83,73.09 C61.1 | v137.91,89.21 C100.2 | v132.6,93.79 C94.2 | v141.45,89.21 C99.2 | v136.14,93.79 C93.2 | v139.56,93.79 C27.2 | v152.93,89.71 C59.1 | v156.34,89.71 C56.1 | v150.28,93.92 C113.1 | v159.13,88.96 C53.1 | v153.82,93.92 C112.1 | v157.36,93.92 C111.1 | v171.99,94.04 171.99,94.44 171.67,94.76 C118.2 | C119.2 183.58,102.3 v183.58,101.98 | v176.18,61.91 176.18,61.84 176.58,61.32 C7.2 | v62.61,84.83 IC4.2 | v26.41,86.26 26.41,85.55 26.18,85.31 Q2.2 | IC11.3 45.31,80.39 v45.31,80.07 | v122.3,67.53 122.3,67.29 121.51,67.29 Q3.2 | v124.05,68.96 124.05,69.2 124.44,69.59 Q10.2 | v161.99,87.38 161.99,86.58 Q16.2 | v161.99,92.45 161.99,91.66 Q14.2
  Top 0.203: v168.34,88.96 168.34,89.44 167.7,89.44 Q15.2 | v167.07,97.22 167.07,97.06 166.59,96.58 Q13.2 | v93.25,68.48 92.53,68.48 C3.2 | v179.45,48.01 179.45,47.29 C2.2 | v174.05,94.04 174.05,94.68 C116.2 | v183.74,99.76 C117.2 | v177.01,62.67 177.01,62.98 176.78,63.34 C4.2 | v104.52,68.33 104.52,69.2 U1.3 | v126.9,62.13 126.9,62.77 126.11,62.77 D7.A | v34.99,83.72 34.99,82.93 34.67,82.61 OSC1.2 | v22.92,95.79 22.92,96.5 22.53,96.9 MOD1.P$1 | v64.2,90.2 64.72,89.76 64.91,90.55 C109.2 | C114.2 55.69,96.54 56.37,97.5 | 63.23,96.47 C115.2 | 64.51,100.58 C110.2 | v162.94,73.09 164.21,73.09 IC12.15 | IC8.4 60.39,74.67 v60.39,74.2 | v74.64,86.74 IC5.4 | v80.98,86.74 IC6.4 | v108.17,62.61 106.98,62.61 IC10.3 | v87.33,86.74 IC7.4 | v93.06,85.49 IC9.4 | v139.19,25.7 140.24,25.62 Q8.3 | v139.19,38.24 140.16,38.23 Q9.3 | v139.19,50.63 140.24,50.62 Q5.3 | v139.26,63.32 140.16,63.23 Q7.3 | v139.19,75.63 140.16,75.62 Q6.3 | v167.23,45.62 167.23,46.97 168.73,48.48 IC1.4
  Top 0.254: v35.78,67.85 35.75,67.88 IC13.10 | v40.86,66.74 40.87,66.75 IC13.99 | v39.75,54.83 IC13.74 | v27.68,61.82 27.62,61.75 IC13.37 | v27.68,66.74 v27.67,66.75 IC13.27 | v30.7,67.85 30.75,67.9 IC13.20 | Q11.3 139.51,13.44 | 132.8,14.38 R36.2
  Top 0.61: v89.6,71.66 89.58,71.64 IC3.2
  Route2 0.203: JP6.20 JP6.18 JP6.16 JP6.14 JP6.12 JP6.10 JP6.8 JP6.6 JP6.4 JP6.2 75.31,101.98 v75.31,100.63 | JP5.2 JP5.4 JP5.6 JP5.8 JP5.10 143.97,101.98 | 143.97,101.98 JP5.12 JP5.14 | JP8.4 JP8.6 JP8.8 JP8.10 JP8.12 | 154.05,101.98 JP4.4 JP4.6 | 154.05,101.98 JP4.2 | v154.05,100.63 154.05,101.98 | 146.59,100.38 143.97,101.98
  AGND$ 0.203: v154.05,100.63 154.05,100.52 | 103.25,100.63 103.25,100.52 | 146.59,100.38 143.97,100.52 | v75.31,100.63 75.31,100.52
  other vias: 102.84,92.26 97.57,93.89 64.17,89.44 62.61,86.42 61.02,79.75 38.84,47.69 40.42,47.69 43.05,47.69 44.64,47.69 46.23,47.69 23.72,53.72 23.72,52.13 19.34,57.21 19.34,54.83 21.18,67.69 21.18,65.31 25.62,74.83 27.21,74.83 31.55,74.83 34.41,74.96 36.25,74.96 37.94,74.98 45.31,70.23 45.31,67.85 49.27,66.74 34.03,83.72 35.62,85.15 46.78,77.23 45.78,83.41 45.31,80.87 50.07,81.98 45.78,84.83 25.62,86.26 25.46,87.53 21.81,95.79 161.35,73.88 174.62,69.98 175.45,78.87 176.27,62.67 177.01,61.91 178.81,48.96 178.66,48.01 180.24,48.01 165.64,51.5 166.43,51.5 167.23,51.5 165.64,45.62 166.43,45.62 165.64,50.7 165.64,49.91 165.64,49.12 165.64,48.01 165.64,47.21 165.64,46.42 89.6,70.07 91.98,70.86 93.25,67.69 93.25,69.28 87.38,70.23 134.05,76.1 134.05,75.15 123.09,68.96 122.3,66.74 126.9,63.56 99.28,58.64 110.22,75.22 110.22,74.43 104.92,76.67 14.44,96.38 14.44,95.59 58.01,73.72 183.58,102.77 183.74,100.55 183.74,98.96 174.85,94.04 173.26,94.04 171.19,94.04 8,118 13,118 18,118 23,118 28,118 33,118 38,118 48,118 53,118 58,118 63,118 68,118 73,118 78,118 83,118 88,118 8,113 3,113 3,108 3,103 3,98 8,108 8,103 8,98 8,93 8,88 3,88 3,83 8,83 18,113 43,113 48,113 53,113 58,113 63,113 68,113 73,113 78,113 83,113 88,113 88,108 83,108 78,108 72.75,108 68.6,108 58.75,108 53.67,108 48,108 43,108 38,108 23,103 28,103 33,103 43,103 48,103 52.1,103 13,98 13,93 18,98 18,93 52.17,98 53,88 38,88 3,78 3,73 3,68 3,58 3,53 3,48 3,43 8,78 8,73 8,68 8,53 8,48 8,43 15.5,83 18,80.5 20.5,78 23,80.5 30.5,83 28,80.5 25.5,78 43,83 40.5,88 48,88 50.5,90.5 55.5,90.5 68,85.5 93,118 98,118 103,118 108,118 113,118 123,118 128,118 133,118 138,118 143,118 148,118 153,118 158,118 163,118 168,118 173,118 178,118 93,113 98,113 103,113 108,113 113,113 118,113 123,113 128,113 133,113 138,113 143,113 148,113 153,113 158,113 163,113 168,113 173,113 178,113 93,108 98,108 103,108 108,108 113,108 118,108 123,108 128,108 133,108 138,108 143,108 148,108 153,108 158,108 163,108 173,108 178,108 104.88,100.62 100.5,85.5 106.5,85.5 102.53,80.62 115.5,78 118,80.5 120.5,83 114,85.75 128,83 125.5,80.5 123,78 120.5,75.5 118,73 110.5,73 111.5,79.85 110.5,68 115.5,68 128,65.5 128,68 130.5,70.5 135.5,70.5 135.5,73 138,73 138,78 140.5,82.3 140.43,69.5 148.15,59.25 136.72,59.55 93,63 95.5,63 183,118 188,118 183,113 183,108 188,108 193,108 193,113 188,103 193,103 193,98 188,98 188,93 183,93 183,88 188,88 183,83 188,83 193,83 193,78 188,78 183,78 183,73 188,73 193,73 193,68 188,68 183,68 178,68 178,73 178,78 175.5,88 168,68 163,68 163,63 168,63 65.5,70.5 68,65.5 73,65.5 78,65.5 80.5,63 83,65.5 85.5,63 88,65.5 70.5,63 70.5,58 78.62,58.5 80.5,58 62.38,57.12 58.88,63.88 71.5,70.5 76.5,70 82.5,70 77.5,72 84.5,72 77.5,74 84.5,74 80.5,75 51.5,67 53.5,67 60.5,53 67.12,53 78,53 78.38,50.25 82.38,50.25 88,50.5 93,50.5 95.5,50.5 100.5,50.5 100.5,47.5 90.5,48 50.5,48 55.5,48 60.5,48 65.5,48 70.5,48 78.62,48 83.75,48 73.12,52.88 35.5,88 43,80.5 43,78 25,90 28,90 31,90 33,89 38,90 41,90 44,90 42,88 46.5,87.5 44,84.5 38.5,80.5 32.5,81.5 29.5,82 29.5,86 25.5,84.5 37,66 38.5,66 18,60 16,60 17,57.5 18,56 21,53.5 18.5,66 19,73.5 18.5,71 36,51.5 36,48 32.38,47.5 29.5,47.5 26.18,46.84 16,44.5 22,45.25 26.5,45 32.12,44.5 34.5,44.5 48.32,50.46 55.74,50.14 60.02,50.14 63.83,50.14 68.6,49.98 61.13,54.75 60.6,63.9 58.59,57.29 47.04,59.35 51.29,57.45 54.31,56.81 54.31,53.79 46.85,54.43 49.55,53.16 58.74,60.7 33.08,63.88 34.51,62.77 38.64,62.77 33.36,60.11 3,38 3,28 3,23 3,18 3,13 3,8 8,8 8,3 13,3 18,3 23,3 33,3 28,3 38,3 48,3 53,3 58,3 63,3 68,3 73,3 73,8 68,8 63,8 58,8 53,8 48,8 43,8 38,8 33,8 28,8 23,8 18,8 13,8 8,13 8,18 8,23 13,18 18,13 13,33 13,28 18,33 18,38 23,38 27.75,38 39.75,37.88 43,38 48,38 53,38 58,38 63,38 68,38 78,38 67,35.38 68,33 63,33 58,33 53,33 48,33 43,33 39,33 27.75,33 23,33 18,28 23,28 43,28 48,28 53,28 58,28 63,28 68,28 78,18 73,18 68,23 63,23 58,23 54.75,22.5 33.25,23.38 28,23.5 23,23 18,23 23,18 28,18 33,18 38,18 43,18 48,18 53,18 58,18 63,18 68,18 78,13 73,13 68,13 63,13 58,13 53,13 48,13 83,38 83,18 83,13 83,8 83,3 88,3 88,8 88,13 88,18 88,23 92,32.88 94.88,39.12 93,28 93,23 93,18 93,13 93,8 93,3 98,3 98,8 103,3 103,8 103,13 103,18 103,23 103,33 103,38 103,43 108,43 108,38 108,33 108,23 108,18 108,13 108,8 108,3 113,3 113,8 113,13 113,18 113,23 113,33 113,38 113,43 118,43 123,43 118,38 123,38 123,33 118,33 118,23 123,23 128,23 133,23 138,23 147,22.65 128,18 123,18 118,18 118,13 123,13 128,13 133,13 138.18,13 138,8 133,8 128,8 123,8 123,3 128,3 133,3 138,3 143,3 148,3 148,8 143,8 153,3 153,8 153,13 153,18 158,3 163,3 168,3 173,3 178,3 158,8 163,8 168,8 173,8 178,8 158,13 163,13 168,13 158,18 163,18 168,18 173,18 183,3 188,3 183,8 188,8 193,8 193,13 193,18 193,23 193,28 193,38 193,43 193,48 193,53 193,58 188,63 188,58 188,53 188,23 188,18 183,18 183,13 178,23 183,28 183,33 183,38 183,43 158,23 158,28 158,33 158,38 158,43 154.12,52.75 153.38,64.25 163,58 168,58 163,53 163,48 163,43 163,38 163,33 163,28 163,23 168,23 168,28 168,33 168,38 173,38 173,33 173,28 173,23 178,28 178,33 178,38 178,43 173,43 168,43 168,53 173,53 36.26,61.26 35.23,58.01 38,58.01 34.94,39.16 37.56,39.16 34.19,39.16 31.57,39.28 36.73,39.16 32.31,39.28 91.06,83.36 85.56,83.36 79.19,83.49 85.68,26.01 82.18,26.01 78.68,26.01 75.06,26.01 71.56,26.01 143.31,93.79 144.95,89.09 108,100.62 113,100.62 113.12,94.75 67.62,103.1 67.85,98 58.62,98.08 62.9,98.08 139.19,13.48
  pour AGND$ (isolate 0.305, no thermals): 0,124 197,124 197,0 0,0
  pour Top (isolate 0.406, no thermals): -0.02,124.28 196.99,124.28 196.99,-0.33 -0.02,-0.33
  pour Route2 (isolate 0.305, no thermals): 0,124 0,0 197,0 197,124
FSMC0  (via drill 0.3)
  Top 0.203: v33,51.1 33,52.45 33.24,52.69 33.24,53.48 IC13.61
  Route2 0.203: v33,51.1 32.61,51.1 31.73,50.23 25.54,50.23 24.83,49.51 22.92,49.51 14.35,40.94 14.35,38.96 13.32,37.92 DSP1.2
FSMC1  (via drill 0.3)
  Top 0.203: v33.72,52.21 33.72,53.48 IC13.62
  Route2 0.203: v33.72,52.21 33.08,52.21 31.5,50.62 25.38,50.62 24.67,49.91 22.76,49.91 13.32,40.46 DSP1.4
FSMC2  (via drill 0.3)
  Top 0.203: v43,54.51 43.8,55.31 43.8,57.69 42.45,57.77 IC13.81
  Route2 0.203: v43,54.51 41.18,52.69 38.24,52.69 34.19,48.64 25.62,48.64 24.59,47.61 v21.97,47.61 | v20.7,48.88 19.19,48.88 13.32,43 DSP1.6
  Route3 0.305: v20.7,48.88 v21.97,47.61
FSMC3  (via drill 0.3)
  Top 0.203: v40.07,56.74 40.07,58.24 41.97,58.24 IC13.82
  Top 0.305: v34.19,50.7 33.56,50.07 v33.56,49.43
  Route2 0.203: v40.07,56.74 39.19,56.74 34.19,51.74 v34.19,50.7 | v33.56,49.43 25.86,49.43 24.67,48.24 v22.61,48.24 | v21.34,49.51 20.38,49.51 20.14,49.27 17.21,49.27 13.48,45.54 13.32,45.54 DSP1.8
  Route3 0.305: v21.34,49.51 v22.61,48.24
FSMC4  (via drill 0.3)
  Top 0.203: v28.95,57.53 28.95,61.18 26.57,61.18 IC13.38
  Route2 0.203: v28.95,57.53 28.95,56.58 27.61,55.23 27.13,55.23 24.75,52.85 24.75,51.66 24.19,51.1 17.92,51.1 14.91,48.08 13.32,48.08 DSP1.10
FSMC5  (via drill 0.3)
  Top 0.203: v27.68,60.23 27.68,60.7 26.57,60.7 IC13.39
  Route2 0.203: v27.68,60.23 27.68,59.83 28.32,59.2 28.32,57.85 25.62,55.15 20.86,55.15 16.33,50.62 13.32,50.62 DSP1.12
FSMC6  (via drill 0.3)
  Top 0.203: v25.3,60.7 25.78,60.23 26.49,60.23 IC13.40
  Route2 0.203: v25.3,60.7 23.48,58.88 15.46,58.88 13.32,56.74 12.84,56.74 12.21,56.1 12.21,54.2 13.24,53.16 DSP1.14
FSMC7  (via drill 0.3)
  Top 0.203: v25.3,59.75 IC13.41
  Route2 0.203: v25.3,59.75 24.91,59.75 23.64,58.48 16.1,58.48 13.32,55.7 DSP1.16
FSMC8  (via drill 0.3)
  Top 0.203: v28.32,56.9 28.32,59.2 27.05,59.28 IC13.42
  Route2 0.203: v28.32,56.9 27.05,55.62 26.97,55.62 24.35,53.01 24.35,51.81 24.03,51.5 17.76,51.5 15.78,49.51 12.84,49.51 11.81,50.55 11.81,52.05 10.78,53.09 DSP1.13
FSMC9  (via drill 0.3)
  Top 0.203: v22.37,60.78 22.37,60.86 24.19,60.86 24.51,60.55 24.51,59.59 25.07,59.04 25.44,58.72 26.49,58.72 IC13.43 | v14.83,60.7 13.71,61.82 11.81,61.82 11.81,56.74 10.78,55.7 DSP1.15
  Route2 0.203: v22.37,60.78 17.13,60.78 17.05,60.7 v14.83,60.7
FSMC10  (via drill 0.3)
  Top 0.203: v24.51,58.32 24.51,58.24 IC13.44
  Route2 0.203: v23.24,59.59 22.13,59.59 21.81,59.28 11.81,59.28 10.78,58.24 DSP1.17
  Route3 0.203: v23.24,59.59 v24.51,58.32
FSMC11  (via drill 0.3)
  Top 0.203: v27.68,58.56 27.68,57.77 26.57,57.77 IC13.45
  Route2 0.203: v27.68,58.56 27.68,59.28 24.99,61.98 11.97,61.98 10.78,60.78 DSP1.19
FSMC12  (via drill 0.3)
  Top 0.203: v23.88,60.23 23.88,57.29 26.49,57.29 IC13.46
  Top 0.305: v14.59,63.48 v16.73,61.34
  Route2 0.203: v23.88,60.23 22.68,61.42 16.81,61.42 v16.73,61.34 | v14.59,63.48 13.71,64.36 11.81,64.36 10.78,63.32 DSP1.21
FSMC13  (via drill 0.3)
  Top 0.203: v29.85,55.61 30.25,54.25 30.23,53.56 IC13.55
  Route2 0.203: v29.85,55.61 29.86,55.86 29.88,57.5 29.85,58.19 28.49,59.67 28.49,61.97 27.89,62.56 24.56,62.56 22.45,64.67 16.81,64.67 14.59,66.9 11.81,66.9 10.78,65.86 DSP1.23
FSMC14  (via drill 0.3)
  Top 0.203: v30.86,55.23 30.78,55.15 30.78,53.56 IC13.56
  Top 0.305: v27.92,47.61 v27.92,52.29 | v14.91,52.05 v21.02,45.94
  Route2 0.203: v27.92,47.61 25.7,47.61 24.03,45.94 v21.02,45.94 | v14.91,52.05 12.84,52.05 11.81,53.09 11.81,56.1 10.78,57.13 10.3,57.13 9.67,57.77 9.67,67.29 10.7,68.33 DSP1.25
  Route3 0.203: v27.92,52.29 v30.86,55.23
FSMC15  (via drill 0.3)
  Top 0.203: v30.7,52.17 31.26,52.85 31.26,53.48 IC13.57 | v19.83,60.15 15.22,64.75 v15.22,67.93
  Route2 0.203: v30.7,52.17 30.65,52.42 27.84,54.59 v27.45,54.59 | v19.83,60.15 v21.73,60.15 | v15.22,67.93 13.32,69.83 11.81,69.83 10.78,70.86 DSP1.27
  Route3 0.203: v27.45,54.59 24.35,57.69 24.19,57.69 v21.73,60.15
GPIOA11  (via drill 0.3, 0.5)
  Top 0.203: IC13.70 37.75,45.88 v40.88,42.75 | R37.1 127.7,14.43 125.38,16.75 v125.38,29.62 | v93.5,42.75 v99.38,36.88
  Route2 0.203: v40.88,42.75 v93.5,42.75 | v99.38,36.88 124.75,36.88 125.25,36.38 125.25,29.75 v125.38,29.62
GPIOB4
  Top 0.203: R102.2 46.89,61.26 45.94,62.21 42.05,62.21 IC13.90
GPIOB5  (via drill 0.3)
  Top 0.203: v46.89,63.64 46.89,64.67 R103.2 | v43.16,63.24 42.69,62.77 42.05,62.77 IC13.91
  Route2 0.203: v46.89,63.64 43.56,63.64 v43.16,63.24
GPIOB6  (via drill 0.3)
  Top 0.203: v44.43,60.63 v53.96,51.1 | v40.86,62.77 41.34,63.24 41.97,63.24 IC13.92 | 130.95,27.21 R46.1
  Top 0.406: v128.97,28.32 130.95,27.21 | v84.01,51.1 v98.17,28.32
  Route2 0.203: v98.17,28.32 v128.97,28.32 | v53.96,51.1 v84.01,51.1
  Route3 0.203: v44.43,60.63 44.12,60.94 42.69,60.94 v40.86,62.77
GPIOB7  (via drill 0.3)
  Top 0.203: v45.62,63.01 44.75,63.88 42.85,63.88 42.77,63.8 42.53,63.72 IC13.93 | v53.48,62.45 60.88,62.45 61,62.25 73.62,49.62 73.62,38 76.83,34.92 C26.1 R21.1
  Route2 0.203: v45.62,63.01 51.5,63.01 52.05,62.45 v53.48,62.45
GPIOB8  (via drill 0.3)
  Top 0.203: IC13.95 40.5,64.75 40.12,64.38 40.12,62 v40.38,61.75 | v34.5,42.5 34.5,41.73 C21.1
  Top 0.254: R11.2 34.61,35.75 | 35.48,35.85 35.75,36.12 35.75,41.25 35.38,41.62
  Top 0.406: 34.61,35.75 R30.1 35.48,35.85 | 35.38,41.62 34.73,41.62 C21.1
  Route3 0.203: 40.25,61.75 37.12,58.62 37.12,54.75 38.25,53.62 38.25,51.62 33.5,46.88 33.5,43.5 v34.5,42.5
  Route3 0.254: v40.38,61.75 40.25,61.75
GPIOB9
  Top 0.203: IC13.96 42.05,65.23 42.69,65.23 43.64,64.28 45.23,64.28 46.1,63.48 46.58,63.01 51.58,63.01 51.58,60.55 52.37,59.75 62.5,59.75 73.12,49.12 73.12,34.12 73.28,33.97 C25.1 R22.1
GPIOB12  (via drill 0.3)
  Top 0.203: v29.11,45.47 27.29,47.29 27.29,52.61 27.61,52.93 27.68,52.93 28.24,53.48 IC13.51 | v71.12,45.47 71.12,34.05 R23.1 C24.1
  Route2 0.203: v71.12,45.47 v29.11,45.47
GPIOB13  (via drill 0.3)
  Top 0.203: v28.72,55.39 28.72,53.56 IC13.52 | v22.37,63.24 20.94,64.67 20.3,64.67 v20.3,65.71 | v17.21,68.8 14.35,71.66 14.35,74.91 13.32,75.94 DSP1.32
  Route2 0.203: v17.21,68.8 v20.3,65.71
  Route3 0.203: v28.72,55.39 24.51,59.59 24.51,60.7 22.37,62.85 v22.37,63.24
GPIOB14  (via drill 0.3)
  Top 0.203: v29.35,54.67 29.27,54.59 29.27,53.56 IC13.53 | v29.82,63.61 29.27,64.19 29.27,66.81 v28.23,67.85
  Route2 0.203: v29.35,54.67 30.46,54.67 30.54,54.59 31.18,54.59 31.5,54.91 31.5,57.22 29.39,59.46 29.26,59.6 29.32,63.29 v29.82,63.61 | v28.23,67.85 27.05,67.85 25.07,69.83 16.89,69.83 13.32,73.41 DSP1.30
GPIOB15  (via drill 0.3)
  Top 0.203: v29.07,52.17 29.75,52.85 29.75,53.48 IC13.54 | v23.36,56.77 23.38,57.51 23,57.93 17.84,63.09 17.84,73.96 13.32,78.48 DSP1.34
  Route2 0.203: v29.07,52.17 28.88,52.29 27.68,53.48 v27.21,53.48 | v23.36,56.77 v24.35,55.78
  Route3 0.203: v27.21,53.48 25.54,55.15 24.99,55.15 v24.35,55.78
GPIOC4  (via drill 0.3)
  Top 0.203: IC13.33 27.12,63.75 27.5,64 v28.38,64 | v31.38,42.62 31.25,42.62 32,41.88
  Top 0.254: R12.2 32.06,35.83 | R31.1 32.98,35.85 33.25,36.12 33.25,41.12 32.88,41.5 32.02,41.62 | 32,41.88 32,41.73 C22.1
  Top 0.406: 32.06,35.83 R31.1 | 32.02,41.62 C22.1
  Route3 0.203: 29.25,63.12 29.25,61.75 29.5,61.5 30.75,61.5 31.25,61 31.25,57.5 32.88,55.75 32.88,52.38 31.38,50.88 v31.38,42.62
  Route3 0.254: v28.38,64 28.62,63.88 29.25,63.12
GPIOC5  (via drill 0.3)
  Top 0.203: IC13.34 25.5,63.25 | 29.5,41.62 30.12,42.25 30.25,42.62 v30.12,42.62
  Top 0.254: R13.2 29.52,35.83 | R34.1 30.48,35.85 30.75,36.12 30.75,41.12 30.38,41.5 29.66,41.5 | 25.5,63.25 v24.88,63.25
  Top 0.406: 29.52,35.83 R34.1 | 29.66,41.5 C23.1 29.5,41.62
  Route3 0.203: v24.88,63.25 25.38,62.5 26.75,61 30.5,61 30.75,60.75 30.75,57.25 31.88,56 31.88,54.62 30,52.75 30,51.38 30.88,50.5 30.88,43.5 v30.12,42.62
GPIOC9  (via drill 0.3)
  Top 0.203: v35.7,54.67 35.7,53.56 IC13.66 | v19.99,50.07 15.62,54.43 15.62,58.4 13.32,60.7 DSP1.20
  Route2 0.203: v35.7,54.67 34.99,54.67 31.34,51.02 25.22,51.02 24.51,50.31 20.22,50.31 v19.99,50.07
GPIOC10  (via drill 0.3)
  Top 0.203: v40.7,56.1 40.7,56.18 41.34,56.26 IC13.78 | v24.35,48.88 22.61,50.62 v22.61,52.13 | 13.32,58.16 13.32,58.09
  Top 0.305: v17.21,54.75 v19.83,52.13 | 13.32,58.09 v14.98,56.42 | 13.32,58.16 DSP1.18
  Route2 0.203: v40.7,56.1 39.12,56.1 35.07,52.05 35.07,50.62 34.51,50.07 32.29,50.07 32.05,49.83 25.7,49.83 24.75,48.88 v24.35,48.88 | v19.83,52.13 v22.61,52.13 | v17.21,54.75 15.54,56.42 v14.98,56.42
GPIOC11  (via drill 0.3)
  Top 0.203: v43.16,56.9 43.16,56.82 42.61,56.74 IC13.79 | v30.08,62.61 28.56,62.61 v28.56,62.85 | v14.59,65.94 14.35,66.18 14.35,67.29 13.32,68.33 DSP1.26
  Route2 0.203: v43.16,56.9 42.13,56.9 40.38,58.64 33.8,58.64 v30.08,62.61 | v21.18,63.48 17.05,63.48 v14.59,65.94
  Route3 0.203: v28.56,62.85 28.2,62.61 27.41,62.61 26.39,63.93 21.58,63.93 v21.18,63.48
GPIOC12  (via drill 0.3)
  Top 0.203: v40.7,57.37 40.7,57.29 41.5,57.21 IC13.80
  Route2 0.203: v40.7,57.37 34.51,57.37 31.65,60.23 v30.02,60.23 | v23.32,62.85 22.92,62.85 22.68,62.61 13.95,62.61 13.32,63.24 DSP1.22
  Route3 0.203: v30.02,60.23 29.14,59.59 27.37,59.59 24.11,62.85 v23.32,62.85
GPIOC13  (via drill 0.3)
  Top 0.203: IC13.7 37.25,67.5 v37.62,67.12 | v37.12,42.25 37.1,41.62 C15.1
  Top 0.254: R10.2 37.15,35.83 | R115.1 38.1,35.85 38.38,36.12 38.38,41.12 38,41.5 37.15,41.5
  Top 0.406: 37.15,35.83 R115.1 | 37.15,41.5 C15.1 37.12,41.5
  Route3 0.203: v37.62,67.12 36.88,67.12 35.75,66 35.75,64.75 36.12,64.38 36.12,62.75 37.25,61.62 37.25,59.5 36.62,58.88 36.62,54.5 37.75,53.38 37.75,51.75 32.88,46.88 32.88,43 34.25,41.62 36.5,41.62 v37.12,42.25
GPIOC14  (via drill 0.3)
  Top 0.203: v36.65,71.14 36.73,71.18 36.73,69.04 IC13.8 | v39.91,72.14 40.15,72.37 40.15,73.96 v40.12,74.44 | v48.12,74.5 51,71.62 52.38,71.62 54.25,73.5 56.5,73.5 60.38,69.62 75.12,69.62 76.12,68.62 76.12,38.25 77.88,36.5 86.5,36.5 86.88,36.12 86.88,34.22 C92.1 R18.1
  Route2 0.203: v39.91,72.14 v38.56,70.79 | v40.12,74.44 41.42,75.48 47.11,75.48 47.25,75.38 v48.12,74.5
  Route3 0.305: v36.65,71.14 38.08,71.14 v38.56,70.79
GPIOC15  (via drill 0.3)
  Top 0.203: v36.02,70.38 36.26,70.39 36.26,69.04 IC13.9 | v46.88,74.62 50.5,70.88 52.88,70.88 54.75,73 55.88,73 59.88,69.12 74.62,69.12 75.5,68.25 75.5,38 77.62,35.88 83.25,35.88 83.91,35.22 C91.1 R19.1
  Route2 0.203: v43.58,74.82 43.81,75 46.5,75 v46.88,74.62
  Route3 0.203: v36.02,70.38 36.42,70.38 37.45,69.59 38.32,69.59 v43.58,74.82
GPIOD2  (via drill 0.3)
  Top 0.203: v98.17,56.02 92.23,56.02 v91.98,55.62 | v48.4,54.83 44.51,58.72 42.05,58.72 IC13.83 | 130.48,64.91 R45.1
  Top 0.406: v128.33,62.77 130.48,64.91
  Route2 0.203: v128.33,62.77 121.43,62.77 112.06,53.4 100.79,53.4 v98.17,56.02 | v91.98,55.62 57.93,55.62 57.13,54.83 v48.4,54.83
GPIOD3  (via drill 0.3)
  Top 0.203: v40.07,59.28 41.97,59.28 IC13.84 | v30.78,63.72 30.54,63.96 v30.54,66.42
  Route2 0.203: v40.07,59.28 35.23,59.28 v30.78,63.72 | v27.53,68.56 27.53,68.88 27.76,69.12 27.76,69.75 26.89,70.63 23.72,70.63 13.32,81.03 DSP1.36
  Route3 0.203: v30.54,66.42 29.99,66.42 29.11,67.29 29.11,68.17 28.72,68.56 v27.53,68.56
GPIOD13  (via drill 0.3)
  Top 0.203: v37.21,44.83 32.37,49.67 32.37,52.45 32.69,52.77 32.77,53.01 IC13.60
  Top 0.406: v128.99,40.31 R47.1 | v93.65,44.83 v98.17,40.31
  Route2 0.203: v98.17,40.31 v128.99,40.31 | v37.21,44.83 v93.65,44.83
GPIOE0  (via drill 0.3)
  Top 0.203: v45.86,65.78 45.86,65.63 43.88,65.63 43.8,65.71 42.45,65.71 IC13.97 | v55.94,68.33 56.97,68.33 59.04,66.26 v59.04,65.86 | v74.62,66.12 75,65.75 75,37.75 77.38,35.38 79.88,35.38 80.36,34.89 C90.1 R20.1
  Route2 0.203: v45.86,65.78 47.37,65.78 49.91,68.33 v55.94,68.33 | v59.04,65.86 64.87,65.86 64.99,65.99 65.5,66.5 74.25,66.5 v74.62,66.12
GPIOE1  (via drill 0.3)
  Top 0.203: v41.26,77.29 42.21,76.34 v42.21,71.74 | v43.16,66.36 42.69,66.26 42.05,66.26 IC13.98 | 31.73,88.01 R43.1
  Top 0.406: 31.73,88.01 32.77,86.98 v32.77,85.55
  Route2 0.203: v32.77,85.55 33.4,84.91 33.4,83.41 39.51,77.29 v41.26,77.29 | v42.21,71.74 42.21,67.69 v43.16,66.36
GPIOE2  (via drill 0.3)
  Top 0.203: 119.28,64.28 119.4,64.16 v119.36,64.12 | 120.32,63.24 R40.1 | 119.28,66.26 Q3.3 | v40.94,68.33 40.31,68.96 IC13.1 | v65.47,61.34 v57.21,69.59 | v105.95,64.75 v104.6,63.4
  Top 0.406: 119.4,64.16 120.32,63.24 | 119.28,66.26 119.28,64.28
  Route2 0.203: v43.83,66.96 45.62,66.96 46.66,68.25 46.66,68.88 47.37,69.59 v57.21,69.59 | v65.47,61.34 66.1,60.7 101.9,60.7 v104.6,63.4 | v105.95,64.75 114.68,64.75 115.31,64.12 v119.36,64.12
  Route3 0.203: v43.83,66.96 42.85,68.33 v40.94,68.33
GPIOE3  (via drill 0.3)
  Top 0.203: v115.31,63.48 v116.58,64.75 | v99.2,55.94 98.65,55.39 v92.93,55.39 | v43.16,52.45 39.43,56.18 39.43,60.23 39.66,60.58 39.66,65.98 39.43,66.58 39.43,68.01 39.75,68.33 IC13.2 | 130,77.14 R50.1
  Top 0.406: v125.47,72.61 130,77.14
  Route2 0.203: v125.47,72.61 124.44,72.61 v116.58,64.75 | v115.31,63.48 113,61.12 113,57.12 111.82,55.94 v99.2,55.94 | v92.93,55.39 91.5,53.96 58.8,53.96 57.13,52.29 43.32,52.29 v43.16,52.45
GPIOE4  (via drill 0.3)
  Top 0.203: v54.83,71.02 v66.9,58.96 | v45.94,74.36 v49.27,71.02 | v41.58,74.36 40.54,73.33 40.54,70.94 39.27,69.67 39.27,69.04 IC13.3 | 130.48,52.61 R49.1
  Top 0.406: v129.6,51.74 130.48,52.61 | v98.17,51.74 96.34,53.56 v95.79,53.56
  Route2 0.203: v98.17,51.74 v129.6,51.74 | v95.79,53.56 92.3,57.05 68.8,57.05 v66.9,58.96 | v49.27,71.02 v54.83,71.02 | v41.58,74.36 42.25,74.12 45.38,74.12 v45.94,74.36
GPIOE6  (via drill 0.3)
  Top 0.203: v103.33,63.17 v107.07,66.91 | v55.47,72.29 v66.42,61.34 | v41.02,69.44 41,70.75 41.25,71 43.25,71 43.75,71.38 v43.72,72.29 | v38.8,67.37 38.24,67.93 38.24,68.96 IC13.5 | 120.55,69.75 R48.1
  Top 0.406: v119.07,70.86 120.55,69.75
  Route2 0.203: v119.07,70.86 111.03,70.86 v107.07,66.91 | v103.33,63.17 100.95,63.17 99.12,61.34 v66.42,61.34 | v55.47,72.29 52.29,72.29 52.05,72.06 51.42,72.06 50.94,72.53 43.96,72.53 v43.72,72.29 | v38.8,67.37 v41.02,69.44
IMESS  (via drill 0.3)
  Top 0.203: v74.83,73.09 63.56,84.36 63.56,85.47 IC4.1 63.48,85.55 | v22.13,76.82 19.67,74.36 19.67,63.58 21,62.12 23.76,62.09 25.7,62.78 26.08,62.77 26.49,62.77 IC13.35 | v50.78,87.06 v45.07,92.77 | D8.A 112,55.28 v110.69,56.59
  Top 0.406: v63.24,87.06 63.48,86.82 63.48,85.55 | IC4.1 64.97,85.51 R52.2 64.97,85.67 65.5,85.67 65.5,84.33 D19.C
  Route2 0.203: v110.69,56.59 110.62,58 110.12,58.5 106.75,58.5 105.86,59.39 105.86,63.22 95.47,72.85 95.23,73.09 v74.83,73.09 | v22.13,76.82 38.08,92.77 v45.07,92.77 | v63.24,87.06 v50.78,87.06
LDCLIGHT  (via drill 0.3)
  Top 0.203: 17.29,88.01 R25.1
  Top 0.406: v14.03,84.76 17.29,88.01
  Route2 0.203: v14.03,84.76 11.89,84.76 10.78,83.64 DSP1.37
N$1
  Top 0.203: 120.63,71.42 R48.2 | 122.54,71.42 R56.1 122.62,71.5 | 124.44,71.5 Q10.1
  Top 0.406: 122.54,71.42 120.63,71.42 | 122.62,71.5 124.44,71.5
N$2  (via drill 0.3)
  Top 0.203: v130.78,78.01 130.91,74.91 126.75,70.63 Q10.3
  Top 0.406: C102.1 130.83,91.95 v130.75,92.83
  Top 0.61: R14.2 130.83,91.95
  Route2 0.203: v130.78,78.01 130.78,78.95 129.17,80.33 129.17,89.26 130.75,91.22 v130.75,92.83
N$3
  Top 0.406: R24.1 R91.2
N$4
  Top 0.203: D6.A 123.01,57.37 123.01,58.48 121.74,59.75 R35.2 121.74,59.91 122.62,60.78 122.62,62.77 D7.C 122.7,62.85 | 121.51,65.47 121.51,65.39 Q3.1 | 124.28,65.47 R33.2
  Top 0.406: 121.51,65.47 122.7,65.47 | 122.7,65.47 124.28,65.47 | 122.7,65.47 122.7,62.85
N$5
  Top 0.203: R88.1 111.81,57.89 D8.C D17.C
N$6
  Top 0.203: 28,85.31 Q2.1 | 28,87.93 R41.1
  Top 0.406: R43.2 R41.1 | 28,87.93 28,85.31
N$7
  Top 0.203: Q4.1 113.17,47.05 112.5,46.38 R27.2 R28.2
N$8
  Top 0.203: 23.24,83.33 R32.2 23.24,83.17 | 20.54,83.33 Q1.1 | 27.05,83.17 Q2.3
  Top 0.406: 20.54,83.33 23.24,83.33 | 23.24,83.17 27.05,83.17
N$9
  Top 0.203: R102.1 48.64,61.26 50.62,61.26 50.62,61.74 LED1.3
N$10
  Top 0.203: 18.95,88.01 R25.2 | 18.4,84.2 Q1.3
  Top 0.406: 18.95,88.01 18.4,87.45 18.4,84.2
N$11
  Top 0.254: D17.A 114.17,54.3 C120.1 110.38,52 109.12,50.75 109.12,50.45 R42.1
N$12
  Top 0.406: JP8.1 85.06,22.93 87.25,25.12 87.25,26.48 R4.1
N$13
  Top 0.203: 172.78,73.64 C64.1 | 170.4,74.28 IC12.3
  Top 0.305: 172.78,73.64 171.59,74.28 170.4,74.28
N$14  (via drill 0.3, 0.5)
  Top 0.406: v146.95,90.92 147.01,90.92 147.01,90.61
